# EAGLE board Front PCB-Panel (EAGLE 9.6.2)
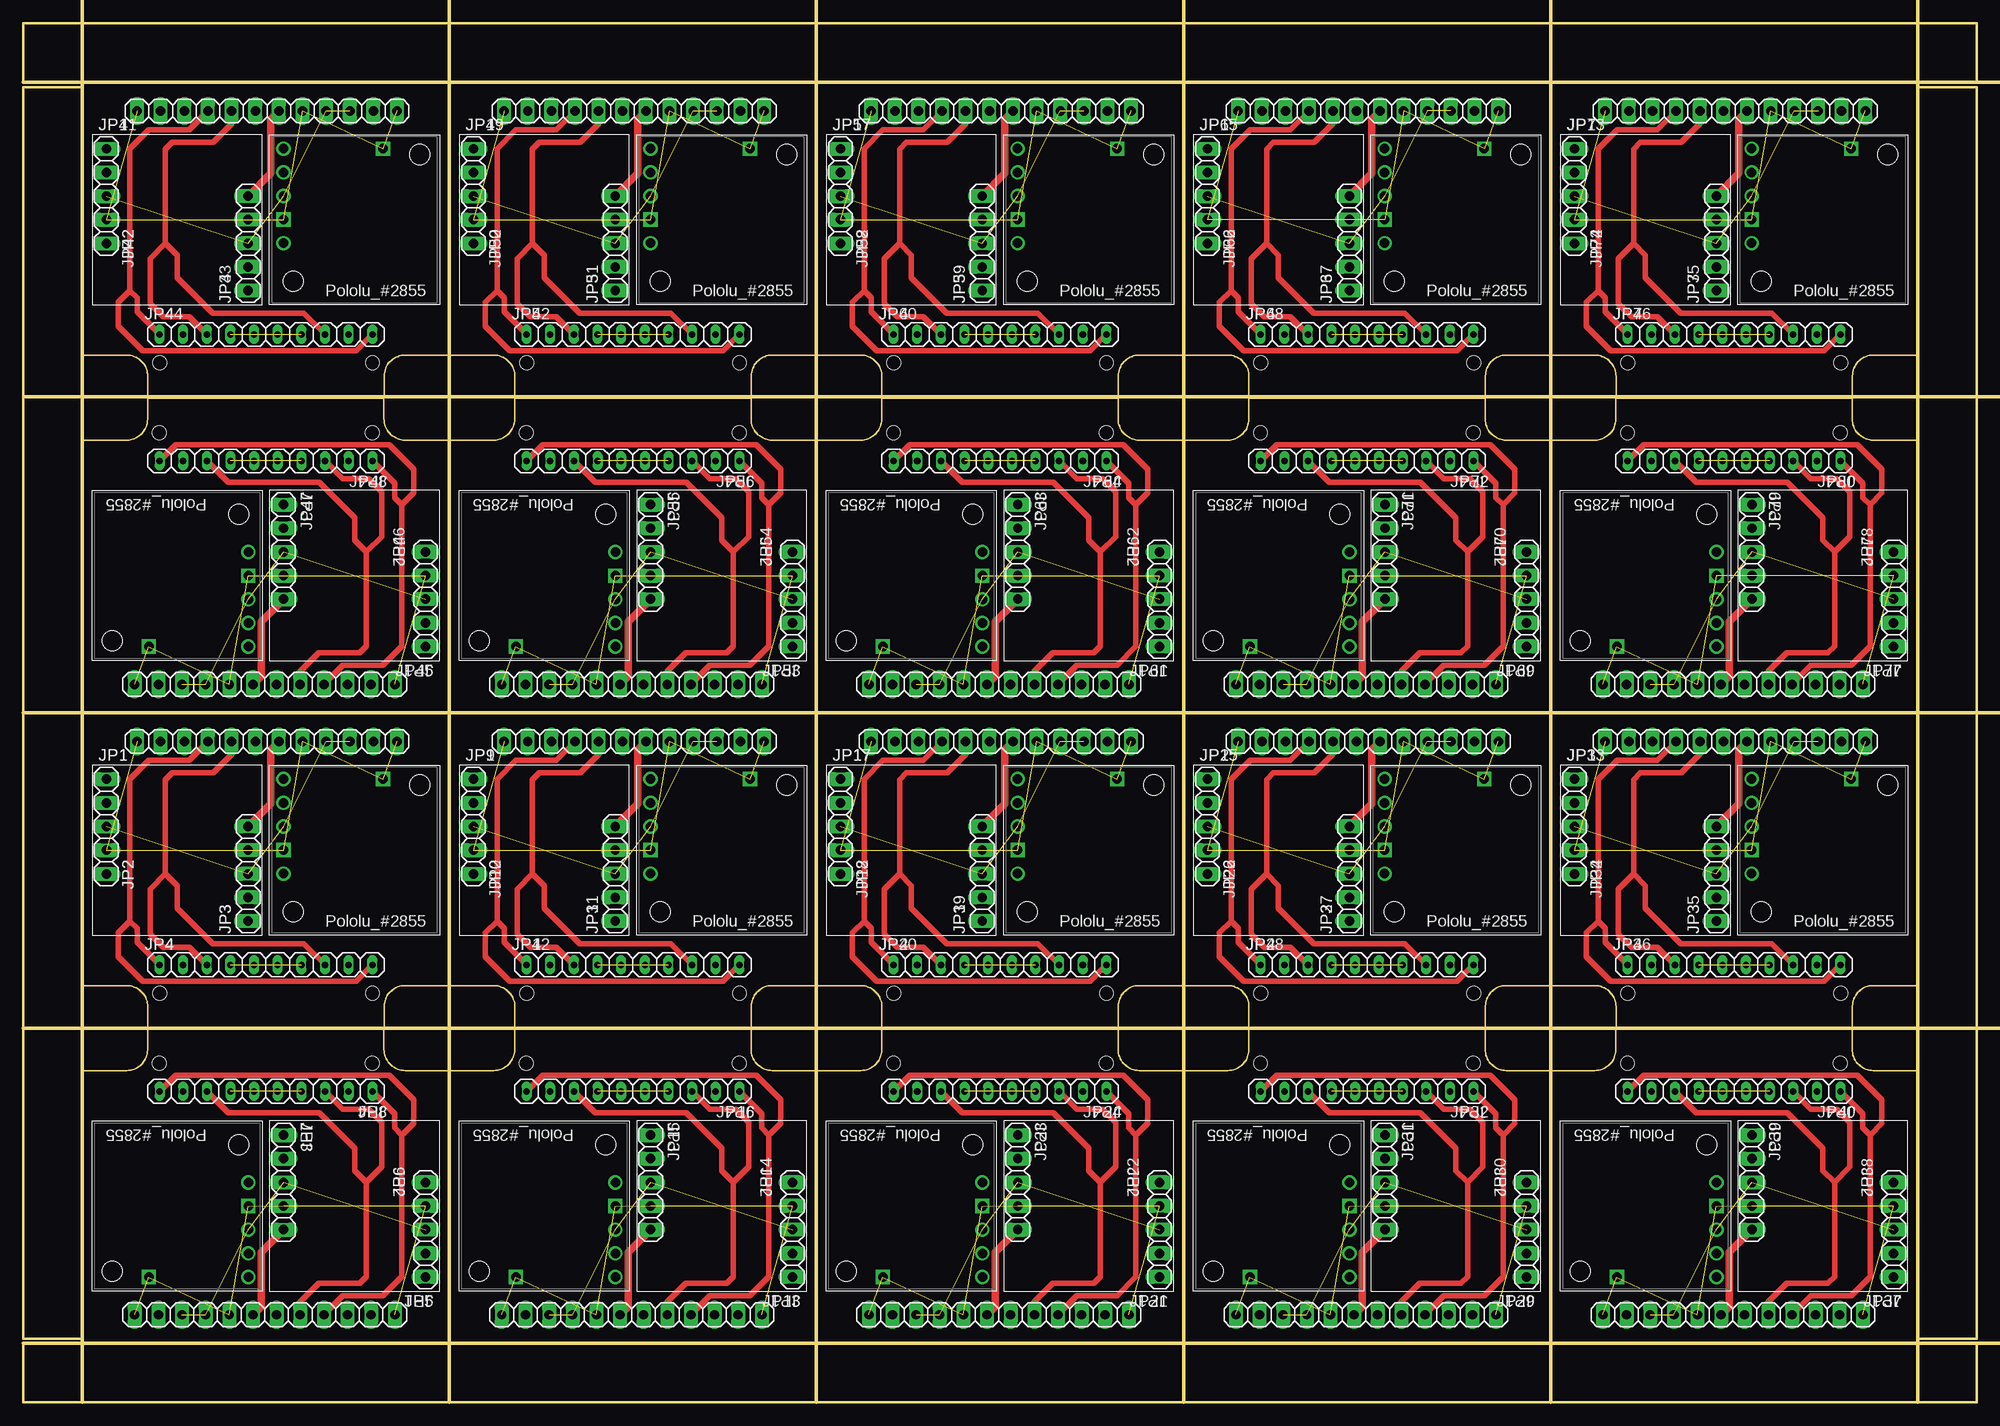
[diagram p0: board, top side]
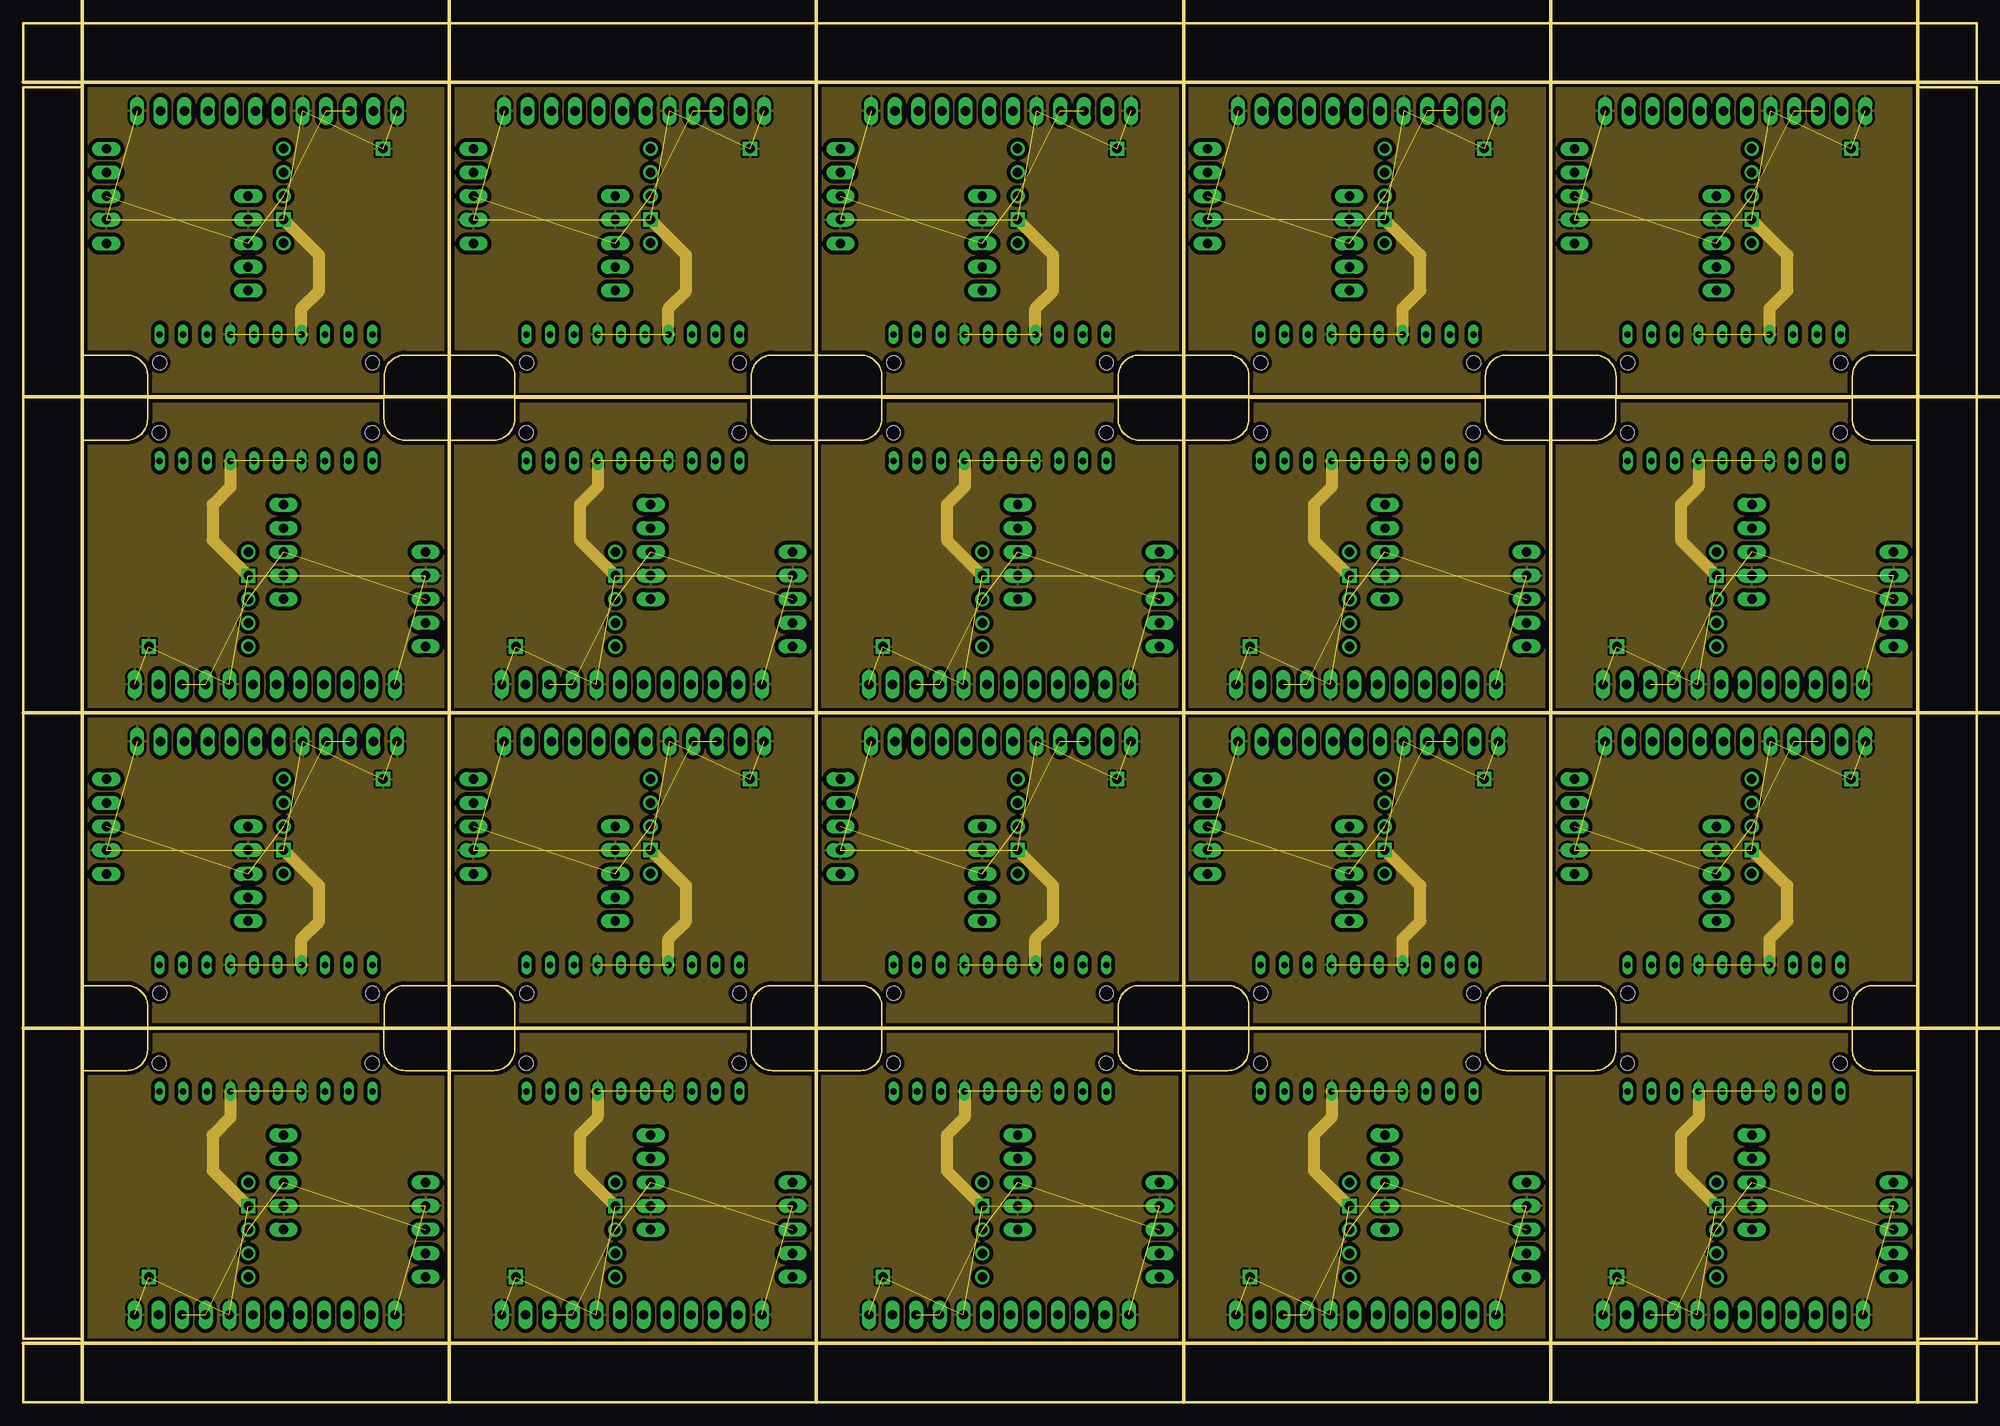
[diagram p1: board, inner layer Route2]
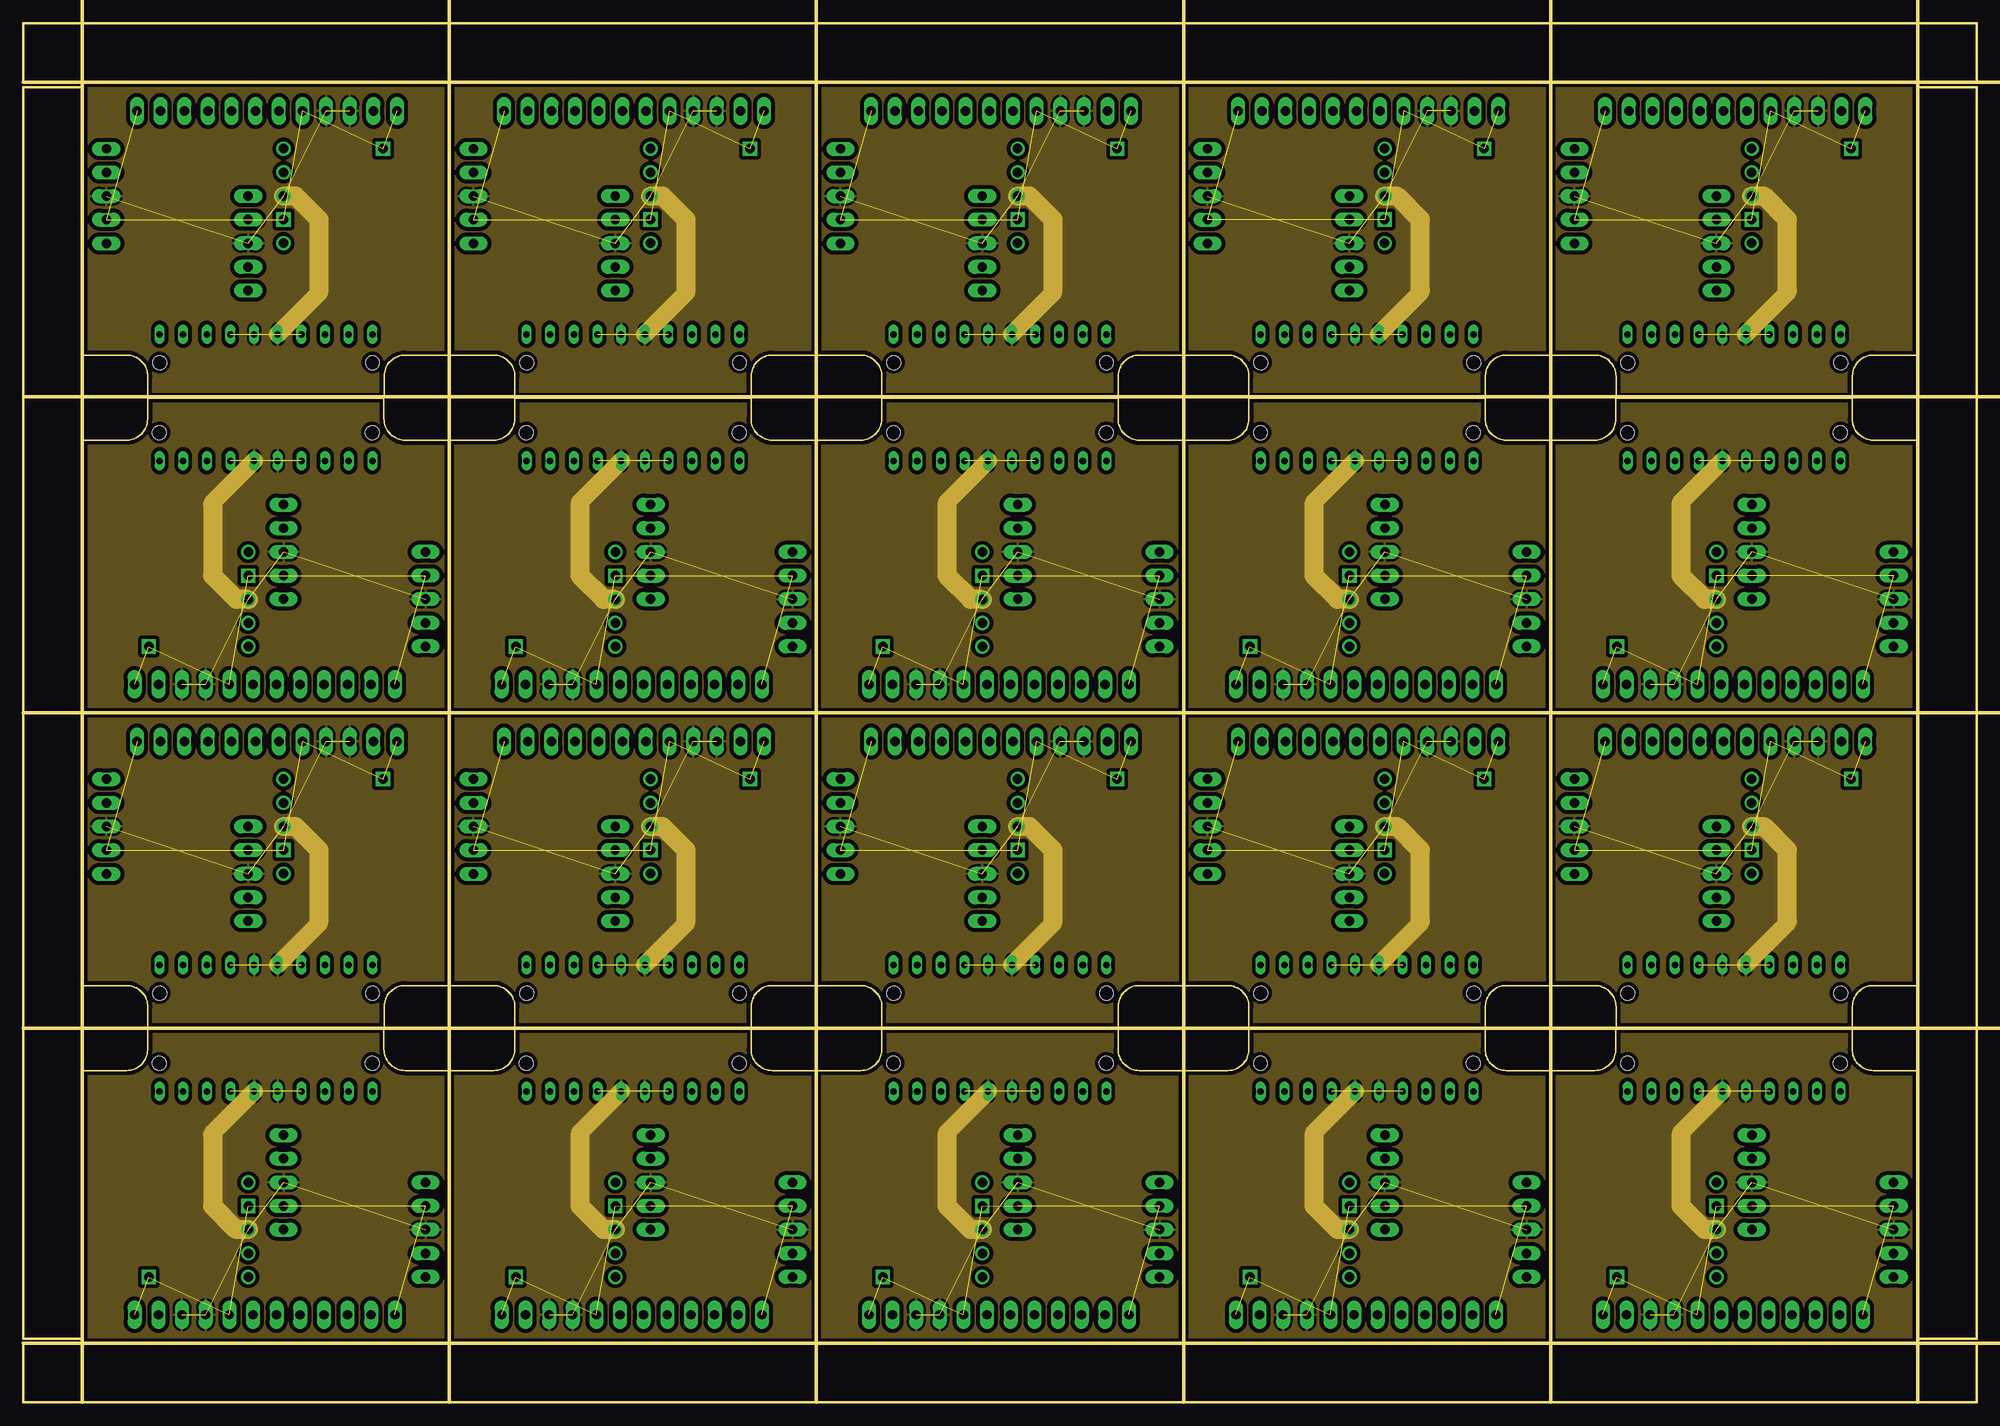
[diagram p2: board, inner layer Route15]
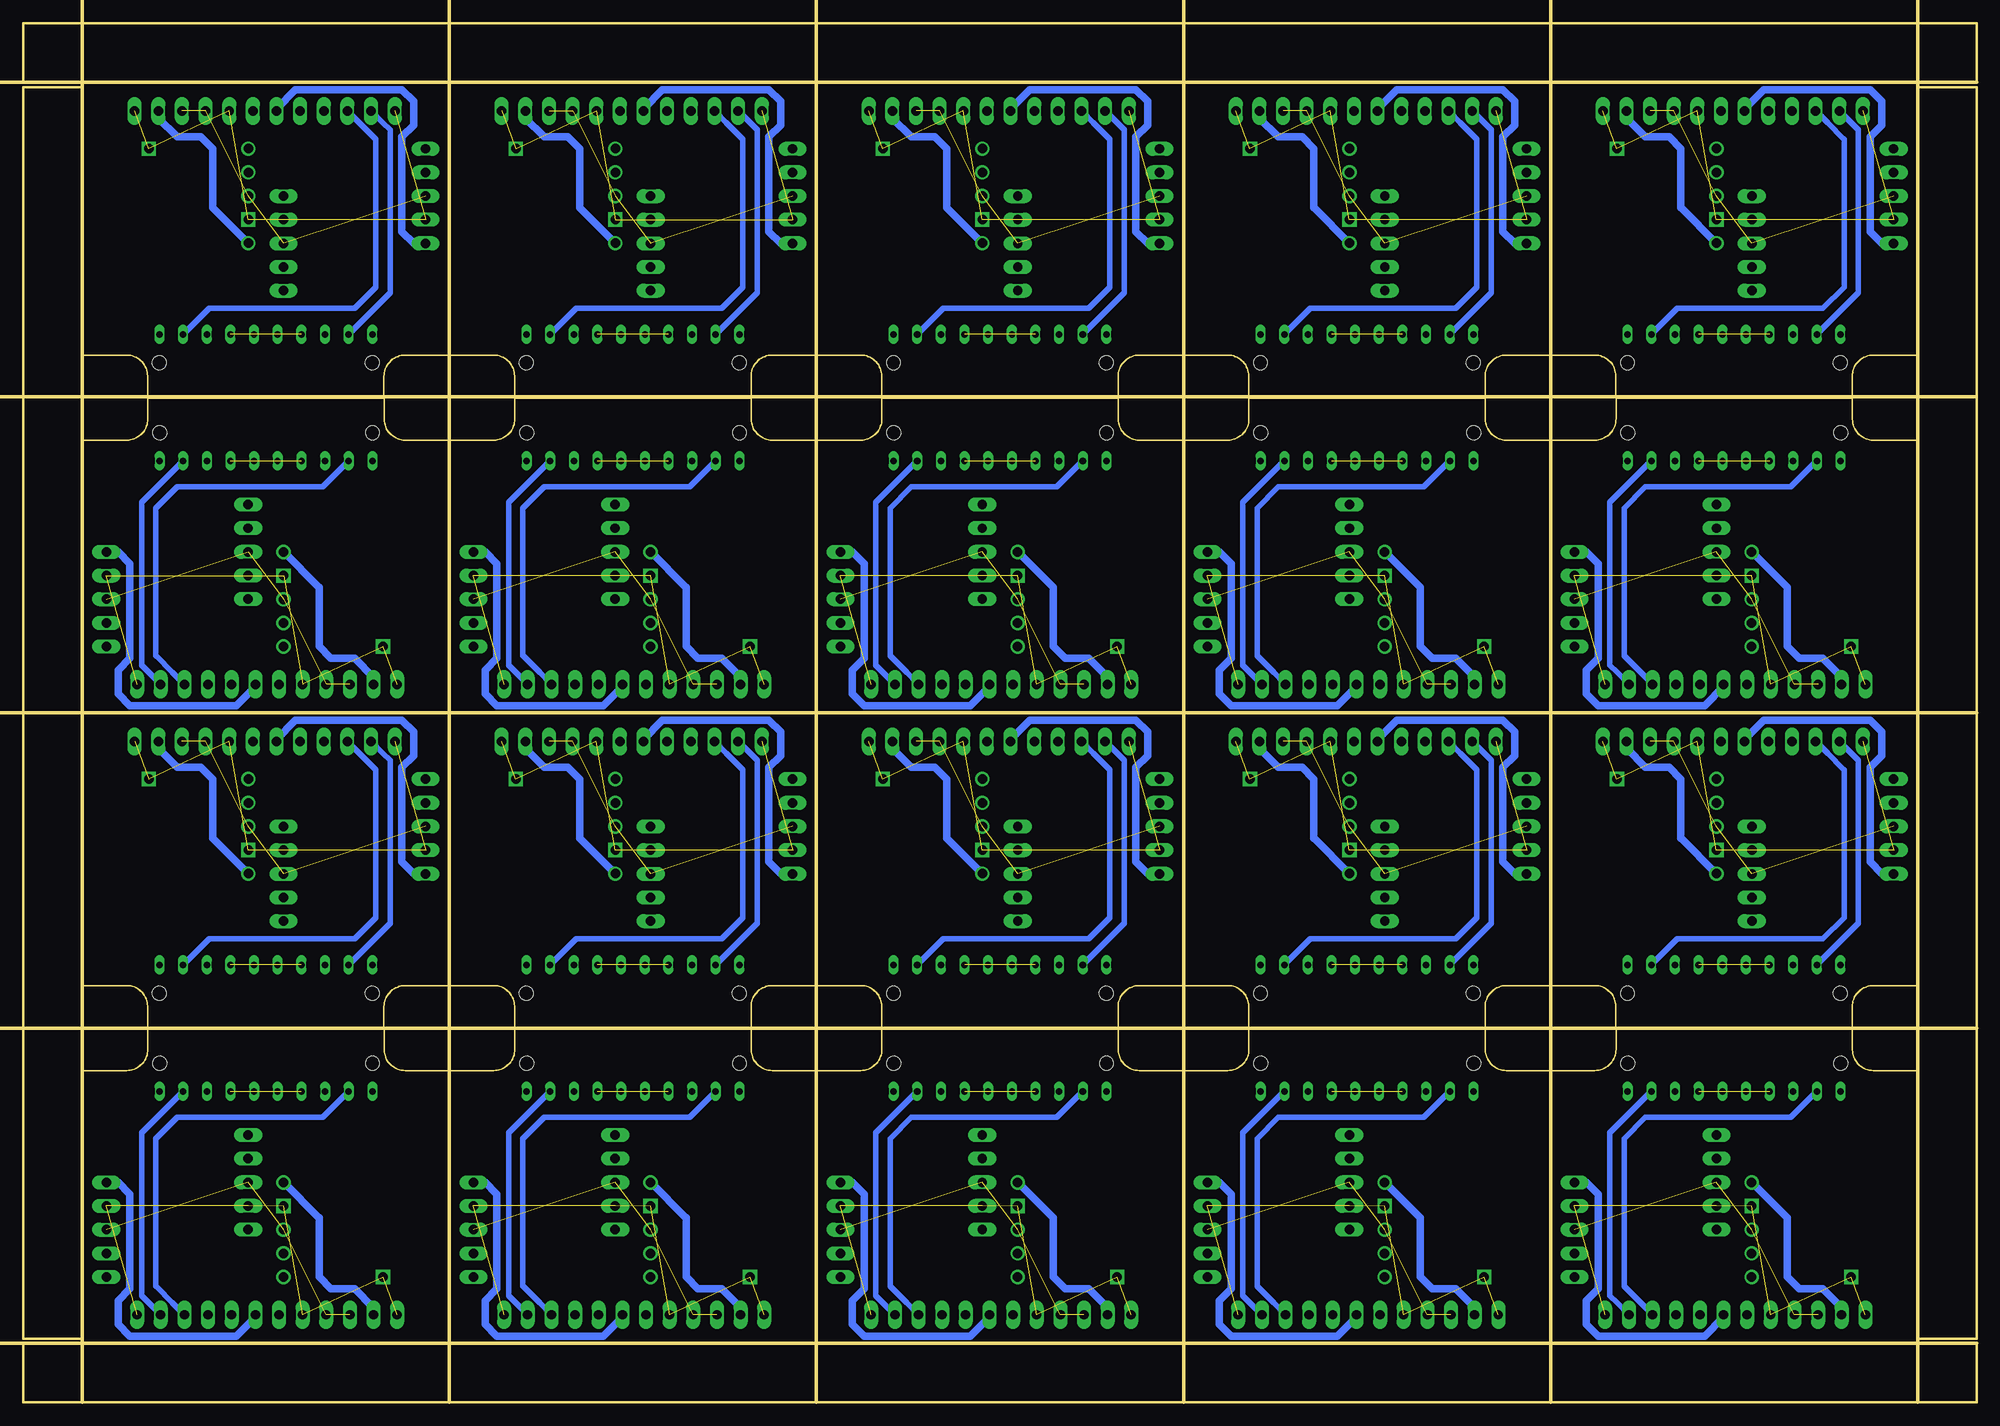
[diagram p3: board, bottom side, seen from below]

Size 209.85 x 148.15 mm. Coordinates in mm from the lower left corner, seen from the top.
Outline: 216 segments
Copper layers 1*2*15*16: Top 0.035mm / dielectric 0.171mm / Route2 0.0178mm / dielectric 44mil / Route15 0.025mm / dielectric 0.171mm / Bottom 0.035mm
Design rules "Front PCB": minimum track width 5mil, minimum drill 0.2mm, track to track 6mil, track to pad 6mil, pad to pad 6mil, via to via 6mil, smd to smd 5mil, copper to edge 0.002540625mm, drill to drill 5mil, minimum pad ring 4mil, minimum via ring 4mil, stop-mask expansion 4mil, vias tented up to drill 0mil, thermal gap 10mil
Holes 1.5 mm at 14.65,43.97 37.51,43.97 37.48,36.45 14.62,36.45 54.08,43.97 76.94,43.97 76.91,36.45 54.05,36.45 93.51,43.97 116.37,43.97 116.34,36.45 93.48,36.45 132.94,43.97 155.8,43.97 155.77,36.45 132.91,36.45 172.37,43.97 195.23,43.97 195.2,36.45 172.34,36.45 14.65,111.7 37.51,111.7 37.48,104.18 14.62,104.18 54.08,111.7 76.94,111.7 76.91,104.18 54.05,104.18 93.51,111.7 116.37,111.7 116.34,104.18 93.48,104.18 132.94,111.7 155.8,111.7 155.77,104.18 132.91,104.18 172.37,111.7 195.23,111.7 195.2,104.18 172.34,104.18
Milling: 11 lines

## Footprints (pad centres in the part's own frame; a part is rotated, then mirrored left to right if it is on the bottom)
POLOLU_D24V22FX = drill 1.02: 1 -7.63,7.63; 2 -7.63,5.09; 3 -7.63,2.55; 5 -7.63,-2.53 | drill 1.02 square: 4 -7.63,0.01; 6 3.06,7.63
1X12 = drill 1.016 long: 1 -13.97,0; 2 -11.43,0; 3 -8.89,0; 4 -6.35,0; 5 -3.81,0; 6 -1.27,0; 7 1.27,0; 8 3.81,0; 9 6.35,0; 10 8.89,0; 11 11.43,0; 12 13.97,0
1X05 = drill 1.016 long: 1 -5.08,0; 2 -2.54,0; 3 0,0; 4 2.54,0; 5 5.08,0
1X10 = drill 0.7 long: P$1 -11.43,0; P$2 -8.89,0; P$3 -6.35,0; P$4 -3.81,0; P$5 -1.27,0; P$6 1.27,0; P$7 3.81,0; P$8 6.35,0; P$9 8.89,0; P$10 11.43,0

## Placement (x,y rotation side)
12V  POLOLU_D24V22FX  [POLOLU_D24V22FX]  35.59,59.33 0 top
12V1  POLOLU_D24V22FX  [POLOLU_D24V22FX]  16.54,21.1 180 top
12V2  POLOLU_D24V22FX  [POLOLU_D24V22FX]  75.02,59.33 0 top
12V3  POLOLU_D24V22FX  [POLOLU_D24V22FX]  55.97,21.1 180 top
12V4  POLOLU_D24V22FX  [POLOLU_D24V22FX]  114.45,59.33 0 top
12V5  POLOLU_D24V22FX  [POLOLU_D24V22FX]  95.4,21.1 180 top
12V6  POLOLU_D24V22FX  [POLOLU_D24V22FX]  153.88,59.33 0 top
12V7  POLOLU_D24V22FX  [POLOLU_D24V22FX]  134.83,21.1 180 top
12V8  POLOLU_D24V22FX  [POLOLU_D24V22FX]  193.31,59.33 0 top
12V9  POLOLU_D24V22FX  [POLOLU_D24V22FX]  174.26,21.1 180 top
12V10  POLOLU_D24V22FX  [POLOLU_D24V22FX]  35.59,127.05 0 top
12V11  POLOLU_D24V22FX  [POLOLU_D24V22FX]  16.54,88.83 180 top
12V12  POLOLU_D24V22FX  [POLOLU_D24V22FX]  75.02,127.05 0 top
12V13  POLOLU_D24V22FX  [POLOLU_D24V22FX]  55.97,88.83 180 top
12V14  POLOLU_D24V22FX  [POLOLU_D24V22FX]  114.45,127.05 0 top
12V15  POLOLU_D24V22FX  [POLOLU_D24V22FX]  95.4,88.83 180 top
12V16  POLOLU_D24V22FX  [POLOLU_D24V22FX]  153.88,127.05 0 top
12V17  POLOLU_D24V22FX  [POLOLU_D24V22FX]  134.83,88.83 180 top
12V18  POLOLU_D24V22FX  [POLOLU_D24V22FX]  193.31,127.05 0 top
12V19  POLOLU_D24V22FX  [POLOLU_D24V22FX]  174.26,88.83 180 top
JP1  [1X12]  26.19,71.01 0 top
JP2  [1X05]  8.92,61.87 270 top
JP3  [1X05]  24.16,56.79 90 top
JP4  1X10  [1X10]  26.07,47.01 0 top
JP5  [1X12]  25.94,9.42 180 top
JP6  [1X05]  43.21,18.56 90 top
JP7  [1X05]  27.97,23.64 270 top
JP8  1X10  [1X10]  26.07,33.42 180 top
JP9  [1X12]  65.62,71.01 0 top
JP10  [1X05]  48.35,61.87 270 top
JP11  [1X05]  63.59,56.79 90 top
JP12  1X10  [1X10]  65.5,47.01 0 top
JP13  [1X12]  65.37,9.42 180 top
JP14  [1X05]  82.64,18.56 90 top
JP15  [1X05]  67.4,23.64 270 top
JP16  1X10  [1X10]  65.5,33.42 180 top
JP17  [1X12]  105.05,71.01 0 top
JP18  [1X05]  87.78,61.87 270 top
JP19  [1X05]  103.02,56.79 90 top
JP20  1X10  [1X10]  104.92,47.01 0 top
JP21  [1X12]  104.8,9.42 180 top
JP22  [1X05]  122.07,18.56 90 top
JP23  [1X05]  106.83,23.64 270 top
JP24  1X10  [1X10]  104.92,33.42 180 top
JP25  [1X12]  144.48,71.01 0 top
JP26  [1X05]  127.21,61.87 270 top
JP27  [1X05]  142.45,56.79 90 top
JP28  1X10  [1X10]  144.36,47.01 0 top
JP29  [1X12]  144.23,9.42 180 top
JP30  [1X05]  161.5,18.56 90 top
JP31  [1X05]  146.26,23.64 270 top
JP32  1X10  [1X10]  144.36,33.42 180 top
JP33  [1X12]  183.91,71.01 0 top
JP34  [1X05]  166.64,61.87 270 top
JP35  [1X05]  181.88,56.79 90 top
JP36  1X10  [1X10]  183.78,47.01 0 top
JP37  [1X12]  183.66,9.42 180 top
JP38  [1X05]  200.93,18.56 90 top
JP39  [1X05]  185.69,23.64 270 top
JP40  1X10  [1X10]  183.78,33.42 180 top
JP41  [1X12]  26.19,138.74 0 top
JP42  [1X05]  8.92,129.59 270 top
JP43  [1X05]  24.16,124.51 90 top
JP44  1X10  [1X10]  26.07,114.73 0 top
JP45  [1X12]  25.94,77.14 180 top
JP46  [1X05]  43.21,86.29 90 top
JP47  [1X05]  27.97,91.37 270 top
JP48  1X10  [1X10]  26.07,101.15 180 top
JP49  [1X12]  65.62,138.74 0 top
JP50  [1X05]  48.35,129.59 270 top
JP51  [1X05]  63.59,124.51 90 top
JP52  1X10  [1X10]  65.5,114.73 0 top
JP53  [1X12]  65.37,77.14 180 top
JP54  [1X05]  82.64,86.29 90 top
JP55  [1X05]  67.4,91.37 270 top
JP56  1X10  [1X10]  65.5,101.15 180 top
JP57  [1X12]  105.05,138.74 0 top
JP58  [1X05]  87.78,129.59 270 top
JP59  [1X05]  103.02,124.51 90 top
JP60  1X10  [1X10]  104.92,114.73 0 top
JP61  [1X12]  104.8,77.14 180 top
JP62  [1X05]  122.07,86.29 90 top
JP63  [1X05]  106.83,91.37 270 top
JP64  1X10  [1X10]  104.92,101.15 180 top
JP65  [1X12]  144.48,138.74 0 top
JP66  [1X05]  127.21,129.59 270 top
JP67  [1X05]  142.45,124.51 90 top
JP68  1X10  [1X10]  144.36,114.73 0 top
JP69  [1X12]  144.23,77.14 180 top
JP70  [1X05]  161.5,86.29 90 top
JP71  [1X05]  146.26,91.37 270 top
JP72  1X10  [1X10]  144.36,101.15 180 top
JP73  [1X12]  183.91,138.74 0 top
JP74  [1X05]  166.64,129.59 270 top
JP75  [1X05]  181.88,124.51 90 top
JP76  1X10  [1X10]  183.78,114.73 0 top
JP77  [1X12]  183.66,77.14 180 top
JP78  [1X05]  200.93,86.29 90 top
JP79  [1X05]  185.69,91.37 270 top
JP80  1X10  [1X10]  183.78,101.15 180 top

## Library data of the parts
12V 12V1-12V19 = POLOLU_D24V22FX
JP1-JP3 JP5-JP7 JP9-JP11 JP13-JP15 JP17-JP19 JP21-JP23 JP25-JP27 JP29-JP31 JP33-JP35 JP37-JP39 JP41-JP43 JP45-JP47 JP49-JP51 JP53-JP55 JP57-JP59 JP61-JP63 JP65-JP67 JP69-JP71 JP73-JP75 JP77-JP79 = pinhead
JP4 JP8 JP12 JP16 JP20 JP24 JP28 JP32 JP36 JP40 JP44 JP48 JP52 JP56 JP60 JP64 JP68 JP72 JP76 JP80 = Pinheads 2.54mm 0.7diameter

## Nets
5V [2A]: JP1.7 JP3.5
5V1 [2A]: JP5.7 JP7.5
5V2 [2A]: JP9.7 JP11.5
5V3 [2A]: JP13.7 JP15.5
5V4 [2A]: JP17.7 JP19.5
5V5 [2A]: JP21.7 JP23.5
5V6 [2A]: JP25.7 JP27.5
5V7 [2A]: JP29.7 JP31.5
5V8 [2A]: JP33.7 JP35.5
5V9 [2A]: JP37.7 JP39.5
5V10 [2A]: JP41.7 JP43.5
5V11 [2A]: JP45.7 JP47.5
5V12 [2A]: JP49.7 JP51.5
5V13 [2A]: JP53.7 JP55.5
5V14 [2A]: JP57.7 JP59.5
5V15 [2A]: JP61.7 JP63.5
5V16 [2A]: JP65.7 JP67.5
5V17 [2A]: JP69.7 JP71.5
5V18 [2A]: JP73.7 JP75.5
5V19 [2A]: JP77.7 JP79.5
6V [1A]: JP1.6 JP2.5
6V1 [1A]: JP5.6 JP6.5
6V2 [1A]: JP9.6 JP10.5
6V3 [1A]: JP13.6 JP14.5
6V4 [1A]: JP17.6 JP18.5
6V5 [1A]: JP21.6 JP22.5
6V6 [1A]: JP25.6 JP26.5
6V7 [1A]: JP29.6 JP30.5
6V8 [1A]: JP33.6 JP34.5
6V9 [1A]: JP37.6 JP38.5
6V10 [1A]: JP41.6 JP42.5
6V11 [1A]: JP45.6 JP46.5
6V12 [1A]: JP49.6 JP50.5
6V13 [1A]: JP53.6 JP54.5
6V14 [1A]: JP57.6 JP58.5
6V15 [1A]: JP61.6 JP62.5
6V16 [1A]: JP65.6 JP66.5
6V17 [1A]: JP69.6 JP70.5
6V18 [1A]: JP73.6 JP74.5
6V19 [1A]: JP77.6 JP78.5
12V [1A]: 12V.5 JP1.11
12V1 [1A]: 12V1.5 JP5.11
12V2 [1A]: 12V2.5 JP9.11
12V3 [1A]: 12V3.5 JP13.11
12V4 [1A]: 12V4.5 JP17.11
12V5 [1A]: 12V5.5 JP21.11
12V6 [1A]: 12V6.5 JP25.11
12V7 [1A]: 12V7.5 JP29.11
12V8 [1A]: 12V8.5 JP33.11
12V9 [1A]: 12V9.5 JP37.11
12V10 [1A]: 12V10.5 JP41.11
12V11 [1A]: 12V11.5 JP45.11
12V12 [1A]: 12V12.5 JP49.11
12V13 [1A]: 12V13.5 JP53.11
12V14 [1A]: 12V14.5 JP57.11
12V15 [1A]: 12V15.5 JP61.11
12V16 [1A]: 12V16.5 JP65.11
12V17 [1A]: 12V17.5 JP69.11
12V18 [1A]: 12V18.5 JP73.11
12V19 [1A]: 12V19.5 JP77.11
24V [3A]: 12V.3 JP1.9 JP1.10 JP2.3 JP3.3 JP4.P$5 JP4.P$6
24V1 [3A]: 12V1.3 JP5.9 JP5.10 JP6.3 JP7.3 JP8.P$5 JP8.P$6
24V2 [3A]: 12V2.3 JP9.9 JP9.10 JP10.3 JP11.3 JP12.P$5 JP12.P$6
24V3 [3A]: 12V3.3 JP13.9 JP13.10 JP14.3 JP15.3 JP16.P$5 JP16.P$6
24V4 [3A]: 12V4.3 JP17.9 JP17.10 JP18.3 JP19.3 JP20.P$5 JP20.P$6
24V5 [3A]: 12V5.3 JP21.9 JP21.10 JP22.3 JP23.3 JP24.P$5 JP24.P$6
24V6 [3A]: 12V6.3 JP25.9 JP25.10 JP26.3 JP27.3 JP28.P$5 JP28.P$6
24V7 [3A]: 12V7.3 JP29.9 JP29.10 JP30.3 JP31.3 JP32.P$5 JP32.P$6
24V8 [3A]: 12V8.3 JP33.9 JP33.10 JP34.3 JP35.3 JP36.P$5 JP36.P$6
24V9 [3A]: 12V9.3 JP37.9 JP37.10 JP38.3 JP39.3 JP40.P$5 JP40.P$6
24V10 [3A]: 12V10.3 JP41.9 JP41.10 JP42.3 JP43.3 JP44.P$5 JP44.P$6
24V11 [3A]: 12V11.3 JP45.9 JP45.10 JP46.3 JP47.3 JP48.P$5 JP48.P$6
24V12 [3A]: 12V12.3 JP49.9 JP49.10 JP50.3 JP51.3 JP52.P$5 JP52.P$6
24V13 [3A]: 12V13.3 JP53.9 JP53.10 JP54.3 JP55.3 JP56.P$5 JP56.P$6
24V14 [3A]: 12V14.3 JP57.9 JP57.10 JP58.3 JP59.3 JP60.P$5 JP60.P$6
24V15 [3A]: 12V15.3 JP61.9 JP61.10 JP62.3 JP63.3 JP64.P$5 JP64.P$6
24V16 [3A]: 12V16.3 JP65.9 JP65.10 JP66.3 JP67.3 JP68.P$5 JP68.P$6
24V17 [3A]: 12V17.3 JP69.9 JP69.10 JP70.3 JP71.3 JP72.P$5 JP72.P$6
24V18 [3A]: 12V18.3 JP73.9 JP73.10 JP74.3 JP75.3 JP76.P$5 JP76.P$6
24V19 [3A]: 12V19.3 JP77.9 JP77.10 JP78.3 JP79.3 JP80.P$5 JP80.P$6
DIR#1: JP1.2 JP4.P$2
DIR#2: JP1.3 JP4.P$9
DIR#3: JP5.2 JP8.P$2
DIR#4: JP5.3 JP8.P$9
DIR#5: JP9.2 JP12.P$2
DIR#6: JP9.3 JP12.P$9
DIR#7: JP13.2 JP16.P$2
DIR#8: JP13.3 JP16.P$9
DIR#9: JP17.2 JP20.P$2
DIR#10: JP17.3 JP20.P$9
DIR#11: JP21.2 JP24.P$2
DIR#12: JP21.3 JP24.P$9
DIR#13: JP25.2 JP28.P$2
DIR#14: JP25.3 JP28.P$9
DIR#15: JP29.2 JP32.P$2
DIR#16: JP29.3 JP32.P$9
DIR#17: JP33.2 JP36.P$2
DIR#18: JP33.3 JP36.P$9
DIR#19: JP37.2 JP40.P$2
DIR#20: JP37.3 JP40.P$9
DIR#21: JP41.2 JP44.P$2
DIR#22: JP41.3 JP44.P$9
DIR#23: JP45.2 JP48.P$2
DIR#24: JP45.3 JP48.P$9
DIR#25: JP49.2 JP52.P$2
DIR#26: JP49.3 JP52.P$9
DIR#27: JP53.2 JP56.P$2
DIR#28: JP53.3 JP56.P$9
DIR#29: JP57.2 JP60.P$2
DIR#30: JP57.3 JP60.P$9
DIR#31: JP61.2 JP64.P$2
DIR#32: JP61.3 JP64.P$9
DIR#33: JP65.2 JP68.P$2
DIR#34: JP65.3 JP68.P$9
DIR#35: JP69.2 JP72.P$2
DIR#36: JP69.3 JP72.P$9
DIR#37: JP73.2 JP76.P$2
DIR#38: JP73.3 JP76.P$9
DIR#39: JP77.2 JP80.P$2
DIR#40: JP77.3 JP80.P$9
GND: 12V.4 12V.6 JP1.1 JP1.8 JP1.12 JP2.4 JP3.4 JP4.P$4 JP4.P$7
GND1: 12V1.4 12V1.6 JP5.1 JP5.8 JP5.12 JP6.4 JP7.4 JP8.P$4 JP8.P$7
GND2: 12V2.4 12V2.6 JP9.1 JP9.8 JP9.12 JP10.4 JP11.4 JP12.P$4 JP12.P$7
GND3: 12V3.4 12V3.6 JP13.1 JP13.8 JP13.12 JP14.4 JP15.4 JP16.P$4 JP16.P$7
GND4: 12V4.4 12V4.6 JP17.1 JP17.8 JP17.12 JP18.4 JP19.4 JP20.P$4 JP20.P$7
GND5: 12V5.4 12V5.6 JP21.1 JP21.8 JP21.12 JP22.4 JP23.4 JP24.P$4 JP24.P$7
GND6: 12V6.4 12V6.6 JP25.1 JP25.8 JP25.12 JP26.4 JP27.4 JP28.P$4 JP28.P$7
GND7: 12V7.4 12V7.6 JP29.1 JP29.8 JP29.12 JP30.4 JP31.4 JP32.P$4 JP32.P$7
GND8: 12V8.4 12V8.6 JP33.1 JP33.8 JP33.12 JP34.4 JP35.4 JP36.P$4 JP36.P$7
GND9: 12V9.4 12V9.6 JP37.1 JP37.8 JP37.12 JP38.4 JP39.4 JP40.P$4 JP40.P$7
GND10: 12V10.4 12V10.6 JP41.1 JP41.8 JP41.12 JP42.4 JP43.4 JP44.P$4 JP44.P$7
GND11: 12V11.4 12V11.6 JP45.1 JP45.8 JP45.12 JP46.4 JP47.4 JP48.P$4 JP48.P$7
GND12: 12V12.4 12V12.6 JP49.1 JP49.8 JP49.12 JP50.4 JP51.4 JP52.P$4 JP52.P$7
GND13: 12V13.4 12V13.6 JP53.1 JP53.8 JP53.12 JP54.4 JP55.4 JP56.P$4 JP56.P$7
GND14: 12V14.4 12V14.6 JP57.1 JP57.8 JP57.12 JP58.4 JP59.4 JP60.P$4 JP60.P$7
GND15: 12V15.4 12V15.6 JP61.1 JP61.8 JP61.12 JP62.4 JP63.4 JP64.P$4 JP64.P$7
GND16: 12V16.4 12V16.6 JP65.1 JP65.8 JP65.12 JP66.4 JP67.4 JP68.P$4 JP68.P$7
GND17: 12V17.4 12V17.6 JP69.1 JP69.8 JP69.12 JP70.4 JP71.4 JP72.P$4 JP72.P$7
GND18: 12V18.4 12V18.6 JP73.1 JP73.8 JP73.12 JP74.4 JP75.4 JP76.P$4 JP76.P$7
GND19: 12V19.4 12V19.6 JP77.1 JP77.8 JP77.12 JP78.4 JP79.4 JP80.P$4 JP80.P$7
HAIVE_ID: JP1.5 JP4.P$3 JP4.P$8
HAIVE_ID1: JP5.5 JP8.P$3 JP8.P$8
HAIVE_ID2: JP9.5 JP12.P$3 JP12.P$8
HAIVE_ID3: JP13.5 JP16.P$3 JP16.P$8
HAIVE_ID4: JP17.5 JP20.P$3 JP20.P$8
HAIVE_ID5: JP21.5 JP24.P$3 JP24.P$8
HAIVE_ID6: JP25.5 JP28.P$3 JP28.P$8
HAIVE_ID7: JP29.5 JP32.P$3 JP32.P$8
HAIVE_ID8: JP33.5 JP36.P$3 JP36.P$8
HAIVE_ID9: JP37.5 JP40.P$3 JP40.P$8
HAIVE_ID10: JP41.5 JP44.P$3 JP44.P$8
HAIVE_ID11: JP45.5 JP48.P$3 JP48.P$8
HAIVE_ID12: JP49.5 JP52.P$3 JP52.P$8
HAIVE_ID13: JP53.5 JP56.P$3 JP56.P$8
HAIVE_ID14: JP57.5 JP60.P$3 JP60.P$8
HAIVE_ID15: JP61.5 JP64.P$3 JP64.P$8
HAIVE_ID16: JP65.5 JP68.P$3 JP68.P$8
HAIVE_ID17: JP69.5 JP72.P$3 JP72.P$8
HAIVE_ID18: JP73.5 JP76.P$3 JP76.P$8
HAIVE_ID19: JP77.5 JP80.P$3 JP80.P$8
SLOT_ID: JP1.4 JP4.P$1 JP4.P$10
SLOT_ID1: JP5.4 JP8.P$1 JP8.P$10
SLOT_ID2: JP9.4 JP12.P$1 JP12.P$10
SLOT_ID3: JP13.4 JP16.P$1 JP16.P$10
SLOT_ID4: JP17.4 JP20.P$1 JP20.P$10
SLOT_ID5: JP21.4 JP24.P$1 JP24.P$10
SLOT_ID6: JP25.4 JP28.P$1 JP28.P$10
SLOT_ID7: JP29.4 JP32.P$1 JP32.P$10
SLOT_ID8: JP33.4 JP36.P$1 JP36.P$10
SLOT_ID9: JP37.4 JP40.P$1 JP40.P$10
SLOT_ID10: JP41.4 JP44.P$1 JP44.P$10
SLOT_ID11: JP45.4 JP48.P$1 JP48.P$10
SLOT_ID12: JP49.4 JP52.P$1 JP52.P$10
SLOT_ID13: JP53.4 JP56.P$1 JP56.P$10
SLOT_ID14: JP57.4 JP60.P$1 JP60.P$10
SLOT_ID15: JP61.4 JP64.P$1 JP64.P$10
SLOT_ID16: JP65.4 JP68.P$1 JP68.P$10
SLOT_ID17: JP69.4 JP72.P$1 JP72.P$10
SLOT_ID18: JP73.4 JP76.P$1 JP76.P$10
SLOT_ID19: JP77.4 JP80.P$1 JP80.P$10

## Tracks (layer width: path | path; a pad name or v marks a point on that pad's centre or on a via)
5V
  Top 0.813: JP3.5 26.59,64.3 26.59,70.14 JP1.7
5V1
  Top 0.813: JP7.5 25.54,16.13 25.54,10.29 JP5.7
5V2
  Top 0.813: JP11.5 66.02,64.3 66.02,70.14 JP9.7
5V3
  Top 0.813: JP15.5 64.97,16.13 64.97,10.29 JP13.7
5V4
  Top 0.813: JP19.5 105.45,64.3 105.45,70.14 JP17.7
5V5
  Top 0.813: JP23.5 104.4,16.13 104.4,10.29 JP21.7
5V6
  Top 0.813: JP27.5 144.88,64.3 144.88,70.14 JP25.7
5V7
  Top 0.813: JP31.5 143.83,16.13 143.83,10.29 JP29.7
5V8
  Top 0.813: JP35.5 184.31,64.3 184.31,70.14 JP33.7
5V9
  Top 0.813: JP39.5 183.26,16.13 183.26,10.29 JP37.7
5V10
  Top 0.813: JP43.5 26.59,132.02 26.59,137.86 JP41.7
5V11
  Top 0.813: JP47.5 25.54,83.86 25.54,78.02 JP45.7
5V12
  Top 0.813: JP51.5 66.02,132.02 66.02,137.86 JP49.7
5V13
  Top 0.813: JP55.5 64.97,83.86 64.97,78.02 JP53.7
5V14
  Top 0.813: JP59.5 105.45,132.02 105.45,137.86 JP57.7
5V15
  Top 0.813: JP63.5 104.4,83.86 104.4,78.02 JP61.7
5V16
  Top 0.813: JP67.5 144.88,132.02 144.88,137.86 JP65.7
5V17
  Top 0.813: JP71.5 143.83,83.86 143.83,78.02 JP69.7
5V18
  Top 0.813: JP75.5 184.31,132.02 184.31,137.86 JP73.7
5V19
  Top 0.813: JP79.5 183.26,83.86 183.26,78.02 JP77.7
6V
  Bottom 0.813: JP1.6 24.92,71.27 22.89,73.3 11.46,73.3 10.19,72.03 10.19,69.49 11.46,68.22 11.46,58.06 10.19,56.79 JP2.5
6V1
  Bottom 0.813: JP5.6 27.21,9.16 29.24,7.13 40.67,7.13 41.94,8.4 41.94,10.94 40.67,12.21 40.67,22.37 41.94,23.64 JP6.5
6V2
  Bottom 0.813: JP9.6 64.35,71.27 62.32,73.3 50.89,73.3 49.62,72.03 49.62,69.49 50.89,68.22 50.89,58.06 49.62,56.79 JP10.5
6V3
  Bottom 0.813: JP13.6 66.64,9.16 68.67,7.13 80.1,7.13 81.37,8.4 81.37,10.94 80.1,12.21 80.1,22.37 81.37,23.64 JP14.5
6V4
  Bottom 0.813: JP17.6 103.78,71.27 101.75,73.3 90.32,73.3 89.05,72.03 89.05,69.49 90.32,68.22 90.32,58.06 89.05,56.79 JP18.5
6V5
  Bottom 0.813: JP21.6 106.07,9.16 108.1,7.13 119.53,7.13 120.8,8.4 120.8,10.94 119.53,12.21 119.53,22.37 120.8,23.64 JP22.5
6V6
  Bottom 0.813: JP25.6 143.21,71.27 141.18,73.3 129.75,73.3 128.48,72.03 128.48,69.49 129.75,68.22 129.75,58.06 128.48,56.79 JP26.5
6V7
  Bottom 0.813: JP29.6 145.5,9.16 147.53,7.13 158.96,7.13 160.23,8.4 160.23,10.94 158.96,12.21 158.96,22.37 160.23,23.64 JP30.5
6V8
  Bottom 0.813: JP33.6 182.64,71.27 180.61,73.3 169.18,73.3 167.91,72.03 167.91,69.49 169.18,68.22 169.18,58.06 167.91,56.79 JP34.5
6V9
  Bottom 0.813: JP37.6 184.93,9.16 186.96,7.13 198.39,7.13 199.66,8.4 199.66,10.94 198.39,12.21 198.39,22.37 199.66,23.64 JP38.5
6V10
  Bottom 0.813: JP41.6 24.92,138.99 22.89,141.02 11.46,141.02 10.19,139.75 10.19,137.21 11.46,135.94 11.46,125.78 10.19,124.51 JP42.5
6V11
  Bottom 0.813: JP45.6 27.21,76.89 29.24,74.86 40.67,74.86 41.94,76.13 41.94,78.67 40.67,79.94 40.67,90.1 41.94,91.37 JP46.5
6V12
  Bottom 0.813: JP49.6 64.35,138.99 62.32,141.02 50.89,141.02 49.62,139.75 49.62,137.21 50.89,135.94 50.89,125.78 49.62,124.51 JP50.5
6V13
  Bottom 0.813: JP53.6 66.64,76.89 68.67,74.86 80.1,74.86 81.37,76.13 81.37,78.67 80.1,79.94 80.1,90.1 81.37,91.37 JP54.5
6V14
  Bottom 0.813: JP57.6 103.78,138.99 101.75,141.02 90.32,141.02 89.05,139.75 89.05,137.21 90.32,135.94 90.32,125.78 89.05,124.51 JP58.5
6V15
  Bottom 0.813: JP61.6 106.07,76.89 108.1,74.86 119.53,74.86 120.8,76.13 120.8,78.67 119.53,79.94 119.53,90.1 120.8,91.37 JP62.5
6V16
  Bottom 0.813: JP65.6 143.21,138.99 141.18,141.02 129.75,141.02 128.48,139.75 128.48,137.21 129.75,135.94 129.75,125.78 128.48,124.51 JP66.5
6V17
  Bottom 0.813: JP69.6 145.5,76.89 147.53,74.86 158.96,74.86 160.23,76.13 160.23,78.67 158.96,79.94 158.96,90.1 160.23,91.37 JP70.5
6V18
  Bottom 0.813: JP73.6 182.64,138.99 180.61,141.02 169.18,141.02 167.91,139.75 167.91,137.21 169.18,135.94 169.18,125.78 167.91,124.51 JP74.5
6V19
  Bottom 0.813: JP77.6 184.93,76.89 186.96,74.86 198.39,74.86 199.66,76.13 199.66,78.67 198.39,79.94 198.39,90.1 199.66,91.37 JP78.5
12V
  Bottom 0.813: 12V.5 31.76,60.6 31.78,60.6 31.78,66.95 33.05,68.22 35.59,68.22 37.62,70.25 JP1.11
12V1
  Bottom 0.813: 12V1.5 20.37,19.83 20.35,19.83 20.35,13.48 19.08,12.21 16.54,12.21 14.51,10.18 JP5.11
12V2
  Bottom 0.813: 12V2.5 71.19,60.6 71.21,60.6 71.21,66.95 72.48,68.22 75.02,68.22 77.05,70.25 JP9.11
12V3
  Bottom 0.813: 12V3.5 59.8,19.83 59.78,19.83 59.78,13.48 58.51,12.21 55.97,12.21 53.94,10.18 JP13.11
12V4
  Bottom 0.813: 12V4.5 110.62,60.6 110.64,60.6 110.64,66.95 111.91,68.22 114.45,68.22 116.48,70.25 JP17.11
12V5
  Bottom 0.813: 12V5.5 99.23,19.83 99.21,19.83 99.21,13.48 97.94,12.21 95.4,12.21 93.37,10.18 JP21.11
12V6
  Bottom 0.813: 12V6.5 150.05,60.6 150.07,60.6 150.07,66.95 151.34,68.22 153.88,68.22 155.91,70.25 JP25.11
12V7
  Bottom 0.813: 12V7.5 138.66,19.83 138.64,19.83 138.64,13.48 137.37,12.21 134.83,12.21 132.8,10.18 JP29.11
12V8
  Bottom 0.813: 12V8.5 189.48,60.6 189.5,60.6 189.5,66.95 190.77,68.22 193.31,68.22 195.34,70.25 JP33.11
12V9
  Bottom 0.813: 12V9.5 178.09,19.83 178.07,19.83 178.07,13.48 176.8,12.21 174.26,12.21 172.23,10.18 JP37.11
12V10
  Bottom 0.813: 12V10.5 31.76,128.32 31.78,128.32 31.78,134.67 33.05,135.94 35.59,135.94 37.62,137.97 JP41.11
12V11
  Bottom 0.813: 12V11.5 20.37,87.56 20.35,87.56 20.35,81.21 19.08,79.94 16.54,79.94 14.51,77.9 JP45.11
12V12
  Bottom 0.813: 12V12.5 71.19,128.32 71.21,128.32 71.21,134.67 72.48,135.94 75.02,135.94 77.05,137.97 JP49.11
12V13
  Bottom 0.813: 12V13.5 59.8,87.56 59.78,87.56 59.78,81.21 58.51,79.94 55.97,79.94 53.94,77.9 JP53.11
12V14
  Bottom 0.813: 12V14.5 110.62,128.32 110.64,128.32 110.64,134.67 111.91,135.94 114.45,135.94 116.48,137.97 JP57.11
12V15
  Bottom 0.813: 12V15.5 99.23,87.56 99.21,87.56 99.21,81.21 97.94,79.94 95.4,79.94 93.37,77.9 JP61.11
12V16
  Bottom 0.813: 12V16.5 150.05,128.32 150.07,128.32 150.07,134.67 151.34,135.94 153.88,135.94 155.91,137.97 JP65.11
12V17
  Bottom 0.813: 12V17.5 138.66,87.56 138.64,87.56 138.64,81.21 137.37,79.94 134.83,79.94 132.8,77.9 JP69.11
12V18
  Bottom 0.813: 12V18.5 189.48,128.32 189.5,128.32 189.5,134.67 190.77,135.94 193.31,135.94 195.34,137.97 JP73.11
12V19
  Bottom 0.813: 12V19.5 178.09,87.56 178.07,87.56 178.07,81.21 176.8,79.94 174.26,79.94 172.23,77.9 JP77.11
24V  (5 unrouted)
  Route15 1.905: JP4.P$6 31.78,51.45 31.78,51.71
  Route15 2.032: 12V.3 29.23,61.88 31.78,59.33 31.78,51.71
  pour Route15 (isolate 0.406): 6.38,74.06 45.75,74.06 45.75,44.34 41.8,44.34 arc90 39.15,41.68 39.15,40.28 12.98,40.28 12.98,41.68 arc90 10.33,44.34 6.38,44.34
24V1  (5 unrouted)
  Route15 1.905: JP8.P$6 20.35,28.97 20.35,28.72
  Route15 2.032: 12V1.3 22.9,18.55 20.35,21.1 20.35,28.72
  pour Route15 (isolate 0.406): 45.75,6.37 6.38,6.37 6.38,36.09 10.33,36.09 arc90 12.98,38.74 12.98,40.15 39.15,40.15 39.15,38.74 arc90 41.8,36.09 45.75,36.09
24V2  (5 unrouted)
  Route15 1.905: JP12.P$6 71.21,51.45 71.21,51.71
  Route15 2.032: 12V2.3 68.66,61.88 71.21,59.33 71.21,51.71
  pour Route15 (isolate 0.406): 45.81,74.06 85.18,74.06 85.18,44.34 81.24,44.34 arc90 78.58,41.68 78.58,40.28 52.42,40.28 52.42,41.68 arc90 49.76,44.34 45.81,44.34
24V3  (5 unrouted)
  Route15 1.905: JP16.P$6 59.78,28.97 59.78,28.72
  Route15 2.032: 12V3.3 62.33,18.55 59.78,21.1 59.78,28.72
  pour Route15 (isolate 0.406): 85.18,6.37 45.81,6.37 45.81,36.09 49.76,36.09 arc90 52.42,38.74 52.42,40.15 78.58,40.15 78.58,38.74 arc90 81.24,36.09 85.18,36.09
24V4  (5 unrouted)
  Route15 1.905: JP20.P$6 110.64,51.45 110.64,51.71
  Route15 2.032: 12V4.3 108.09,61.88 110.64,59.33 110.64,51.71
  pour Route15 (isolate 0.406): 85.24,74.06 124.61,74.06 124.61,44.34 120.66,44.34 arc90 118.01,41.68 118.01,40.28 91.84,40.28 91.84,41.68 arc90 89.19,44.34 85.24,44.34
24V5  (5 unrouted)
  Route15 1.905: JP24.P$6 99.21,28.97 99.21,28.72
  Route15 2.032: 12V5.3 101.76,18.55 99.21,21.1 99.21,28.72
  pour Route15 (isolate 0.406): 124.61,6.37 85.24,6.37 85.24,36.09 89.19,36.09 arc90 91.84,38.74 91.84,40.15 118.01,40.15 118.01,38.74 arc90 120.66,36.09 124.61,36.09
24V6  (5 unrouted)
  Route15 1.905: JP28.P$6 150.07,51.45 150.07,51.71
  Route15 2.032: 12V6.3 147.52,61.88 150.07,59.33 150.07,51.71
  pour Route15 (isolate 0.406): 124.67,74.06 164.04,74.06 164.04,44.34 160.09,44.34 arc90 157.44,41.68 157.44,40.28 131.27,40.28 131.27,41.68 arc90 128.62,44.34 124.67,44.34
24V7  (5 unrouted)
  Route15 1.905: JP32.P$6 138.64,28.97 138.64,28.72
  Route15 2.032: 12V7.3 141.19,18.55 138.64,21.1 138.64,28.72
  pour Route15 (isolate 0.406): 164.04,6.37 124.67,6.37 124.67,36.09 128.62,36.09 arc90 131.27,38.74 131.27,40.15 157.44,40.15 157.44,38.74 arc90 160.09,36.09 164.04,36.09
24V8  (5 unrouted)
  Route15 1.905: JP36.P$6 189.5,51.45 189.5,51.71
  Route15 2.032: 12V8.3 186.95,61.88 189.5,59.33 189.5,51.71
  pour Route15 (isolate 0.406): 164.1,74.06 203.47,74.06 203.47,44.34 199.52,44.34 arc90 196.87,41.68 196.87,40.28 170.7,40.28 170.7,41.68 arc90 168.05,44.34 164.1,44.34
24V9  (5 unrouted)
  Route15 1.905: JP40.P$6 178.07,28.97 178.07,28.72
  Route15 2.032: 12V9.3 180.62,18.55 178.07,21.1 178.07,28.72
  pour Route15 (isolate 0.406): 203.47,6.37 164.1,6.37 164.1,36.09 168.05,36.09 arc90 170.7,38.74 170.7,40.15 196.87,40.15 196.87,38.74 arc90 199.52,36.09 203.47,36.09
24V10  (5 unrouted)
  Route15 1.905: JP44.P$6 31.78,119.18 31.78,119.43
  Route15 2.032: 12V10.3 29.23,129.6 31.78,127.05 31.78,119.43
  pour Route15 (isolate 0.406): 6.38,141.79 45.75,141.79 45.75,112.07 41.8,112.07 arc90 39.15,109.41 39.15,108 12.98,108 12.98,109.41 arc90 10.33,112.07 6.38,112.07
24V11  (5 unrouted)
  Route15 1.905: JP48.P$6 20.35,96.7 20.35,96.45
  Route15 2.032: 12V11.3 22.9,86.28 20.35,88.83 20.35,96.45
  pour Route15 (isolate 0.406): 45.75,74.09 6.38,74.09 6.38,103.81 10.33,103.81 arc90 12.98,106.47 12.98,107.88 39.15,107.88 39.15,106.47 arc90 41.8,103.81 45.75,103.81
24V12  (5 unrouted)
  Route15 1.905: JP52.P$6 71.21,119.18 71.21,119.43
  Route15 2.032: 12V12.3 68.66,129.6 71.21,127.05 71.21,119.43
  pour Route15 (isolate 0.406): 45.81,141.79 85.18,141.79 85.18,112.07 81.24,112.07 arc90 78.58,109.41 78.58,108 52.42,108 52.42,109.41 arc90 49.76,112.07 45.81,112.07
24V13  (5 unrouted)
  Route15 1.905: JP56.P$6 59.78,96.7 59.78,96.45
  Route15 2.032: 12V13.3 62.33,86.28 59.78,88.83 59.78,96.45
  pour Route15 (isolate 0.406): 85.18,74.09 45.81,74.09 45.81,103.81 49.76,103.81 arc90 52.42,106.47 52.42,107.88 78.58,107.88 78.58,106.47 arc90 81.24,103.81 85.18,103.81
24V14  (5 unrouted)
  Route15 1.905: JP60.P$6 110.64,119.18 110.64,119.43
  Route15 2.032: 12V14.3 108.09,129.6 110.64,127.05 110.64,119.43
  pour Route15 (isolate 0.406): 85.24,141.79 124.61,141.79 124.61,112.07 120.66,112.07 arc90 118.01,109.41 118.01,108 91.84,108 91.84,109.41 arc90 89.19,112.07 85.24,112.07
24V15  (5 unrouted)
  Route15 1.905: JP64.P$6 99.21,96.7 99.21,96.45
  Route15 2.032: 12V15.3 101.76,86.28 99.21,88.83 99.21,96.45
  pour Route15 (isolate 0.406): 124.61,74.09 85.24,74.09 85.24,103.81 89.19,103.81 arc90 91.84,106.47 91.84,107.88 118.01,107.88 118.01,106.47 arc90 120.66,103.81 124.61,103.81
24V16  (5 unrouted)
  Route15 1.905: JP68.P$6 150.07,119.18 150.07,119.43
  Route15 2.032: 12V16.3 147.52,129.6 150.07,127.05 150.07,119.43
  pour Route15 (isolate 0.406): 124.67,141.79 164.04,141.79 164.04,112.07 160.09,112.07 arc90 157.44,109.41 157.44,108 131.27,108 131.27,109.41 arc90 128.62,112.07 124.67,112.07
24V17  (5 unrouted)
  Route15 1.905: JP72.P$6 138.64,96.7 138.64,96.45
  Route15 2.032: 12V17.3 141.19,86.28 138.64,88.83 138.64,96.45
  pour Route15 (isolate 0.406): 164.04,74.09 124.67,74.09 124.67,103.81 128.62,103.81 arc90 131.27,106.47 131.27,107.88 157.44,107.88 157.44,106.47 arc90 160.09,103.81 164.04,103.81
24V18  (5 unrouted)
  Route15 1.905: JP76.P$6 189.5,119.18 189.5,119.43
  Route15 2.032: 12V18.3 186.95,129.6 189.5,127.05 189.5,119.43
  pour Route15 (isolate 0.406): 164.1,141.79 203.47,141.79 203.47,112.07 199.52,112.07 arc90 196.87,109.41 196.87,108 170.7,108 170.7,109.41 arc90 168.05,112.07 164.1,112.07
24V19  (5 unrouted)
  Route15 1.905: JP80.P$6 178.07,96.7 178.07,96.45
  Route15 2.032: 12V19.3 180.62,86.28 178.07,88.83 178.07,96.45
  pour Route15 (isolate 0.406): 203.47,74.09 164.1,74.09 164.1,103.81 168.05,103.81 arc90 170.7,106.47 170.7,107.88 196.87,107.88 196.87,106.47 arc90 199.52,103.81 203.47,103.81
DIR#1
  Bottom 0.61: JP1.2 13.49,69.74 13.49,69.72 12.73,68.97 12.73,51.45 JP4.P$2
DIR#2
  Bottom 0.61: JP1.3 16.03,69.74 16.03,69.72 14.27,67.96 14.25,67.96 14.25,52.09 16.54,49.8 31.78,49.8 32.16,49.8 JP4.P$9
DIR#3
  Bottom 0.61: JP5.2 38.64,10.69 38.64,10.7 39.4,11.46 39.4,28.97 JP8.P$2
DIR#4
  Bottom 0.61: JP5.3 36.1,10.69 36.1,10.7 37.86,12.46 37.88,12.46 37.88,28.34 35.59,30.62 19.97,30.62 JP8.P$9
DIR#5
  Bottom 0.61: JP9.2 52.92,69.74 52.92,69.72 52.16,68.97 52.16,51.45 JP12.P$2
DIR#6
  Bottom 0.61: JP9.3 55.46,69.74 55.46,69.72 53.7,67.96 53.69,67.96 53.69,52.09 55.97,49.8 71.21,49.8 71.59,49.8 JP12.P$9
DIR#7
  Bottom 0.61: JP13.2 78.07,10.69 78.07,10.7 78.83,11.46 78.83,28.97 JP16.P$2
DIR#8
  Bottom 0.61: JP13.3 75.53,10.69 75.53,10.7 77.29,12.46 77.31,12.46 77.31,28.34 75.02,30.62 59.4,30.62 JP16.P$9
DIR#9
  Bottom 0.61: JP17.2 92.35,69.74 92.35,69.72 91.59,68.97 91.59,51.45 JP20.P$2
DIR#10
  Bottom 0.61: JP17.3 94.89,69.74 94.89,69.72 93.13,67.96 93.11,67.96 93.11,52.09 95.4,49.8 110.64,49.8 111.02,49.8 JP20.P$9
DIR#11
  Bottom 0.61: JP21.2 117.5,10.69 117.5,10.7 118.26,11.46 118.26,28.97 JP24.P$2
DIR#12
  Bottom 0.61: JP21.3 114.96,10.69 114.96,10.7 116.72,12.46 116.74,12.46 116.74,28.34 114.45,30.62 98.83,30.62 JP24.P$9
DIR#13
  Bottom 0.61: JP25.2 131.78,69.74 131.78,69.72 131.02,68.97 131.02,51.45 JP28.P$2
DIR#14
  Bottom 0.61: JP25.3 134.32,69.74 134.32,69.72 132.56,67.96 132.54,67.96 132.54,52.09 134.83,49.8 150.07,49.8 150.45,49.8 JP28.P$9
DIR#15
  Bottom 0.61: JP29.2 156.93,10.69 156.93,10.7 157.69,11.46 157.69,28.97 JP32.P$2
DIR#16
  Bottom 0.61: JP29.3 154.39,10.69 154.39,10.7 156.15,12.46 156.17,12.46 156.17,28.34 153.88,30.62 138.26,30.62 JP32.P$9
DIR#17
  Bottom 0.61: JP33.2 171.21,69.74 171.21,69.72 170.45,68.97 170.45,51.45 JP36.P$2
DIR#18
  Bottom 0.61: JP33.3 173.75,69.74 173.75,69.72 171.99,67.96 171.97,67.96 171.97,52.09 174.26,49.8 189.5,49.8 189.88,49.8 JP36.P$9
DIR#19
  Bottom 0.61: JP37.2 196.36,10.69 196.36,10.7 197.12,11.46 197.12,28.97 JP40.P$2
DIR#20
  Bottom 0.61: JP37.3 193.82,10.69 193.82,10.7 195.58,12.46 195.59,12.46 195.59,28.34 193.31,30.62 177.69,30.62 JP40.P$9
DIR#21
  Bottom 0.61: JP41.2 13.49,137.46 13.49,137.45 12.73,136.69 12.73,119.18 JP44.P$2
DIR#22
  Bottom 0.61: JP41.3 16.03,137.46 16.03,137.45 14.27,135.69 14.25,135.69 14.25,119.81 16.54,117.53 31.78,117.53 32.16,117.53 JP44.P$9
DIR#23
  Bottom 0.61: JP45.2 38.64,78.42 38.64,78.43 39.4,79.19 39.4,96.7 JP48.P$2
DIR#24
  Bottom 0.61: JP45.3 36.1,78.42 36.1,78.43 37.86,80.19 37.88,80.19 37.88,96.06 35.59,98.35 19.97,98.35 JP48.P$9
DIR#25
  Bottom 0.61: JP49.2 52.92,137.46 52.92,137.45 52.16,136.69 52.16,119.18 JP52.P$2
DIR#26
  Bottom 0.61: JP49.3 55.46,137.46 55.46,137.45 53.7,135.69 53.69,135.69 53.69,119.81 55.97,117.53 71.21,117.53 71.59,117.53 JP52.P$9
DIR#27
  Bottom 0.61: JP53.2 78.07,78.42 78.07,78.43 78.83,79.19 78.83,96.7 JP56.P$2
DIR#28
  Bottom 0.61: JP53.3 75.53,78.42 75.53,78.43 77.29,80.19 77.31,80.19 77.31,96.06 75.02,98.35 59.4,98.35 JP56.P$9
DIR#29
  Bottom 0.61: JP57.2 92.35,137.46 92.35,137.45 91.59,136.69 91.59,119.18 JP60.P$2
DIR#30
  Bottom 0.61: JP57.3 94.89,137.46 94.89,137.45 93.13,135.69 93.11,135.69 93.11,119.81 95.4,117.53 110.64,117.53 111.02,117.53 JP60.P$9
DIR#31
  Bottom 0.61: JP61.2 117.5,78.42 117.5,78.43 118.26,79.19 118.26,96.7 JP64.P$2
DIR#32
  Bottom 0.61: JP61.3 114.96,78.42 114.96,78.43 116.72,80.19 116.74,80.19 116.74,96.06 114.45,98.35 98.83,98.35 JP64.P$9
DIR#33
  Bottom 0.61: JP65.2 131.78,137.46 131.78,137.45 131.02,136.69 131.02,119.18 JP68.P$2
DIR#34
  Bottom 0.61: JP65.3 134.32,137.46 134.32,137.45 132.56,135.69 132.54,135.69 132.54,119.81 134.83,117.53 150.07,117.53 150.45,117.53 JP68.P$9
DIR#35
  Bottom 0.61: JP69.2 156.93,78.42 156.93,78.43 157.69,79.19 157.69,96.7 JP72.P$2
DIR#36
  Bottom 0.61: JP69.3 154.39,78.42 154.39,78.43 156.15,80.19 156.17,80.19 156.17,96.06 153.88,98.35 138.26,98.35 JP72.P$9
DIR#37
  Bottom 0.61: JP73.2 171.21,137.46 171.21,137.45 170.45,136.69 170.45,119.18 JP76.P$2
DIR#38
  Bottom 0.61: JP73.3 173.75,137.46 173.75,137.45 171.99,135.69 171.97,135.69 171.97,119.81 174.26,117.53 189.5,117.53 189.88,117.53 JP76.P$9
DIR#39
  Bottom 0.61: JP77.2 196.36,78.42 196.36,78.43 197.12,79.19 197.12,96.7 JP80.P$2
DIR#40
  Bottom 0.61: JP77.3 193.82,78.42 193.82,78.43 195.58,80.19 195.59,80.19 195.59,96.06 193.31,98.35 177.69,98.35 JP80.P$9
GND  (7 unrouted)
  Route2 1.27: 12V.4 31.78,55.52 31.78,51.71 29.88,49.8 JP4.P$7
  pour Route2 (isolate 0.406): 6.38,74.06 45.75,74.06 45.75,44.34 42,44.34 arc90 39.02,41.36 39.02,40.28 13.24,40.28 13.24,41.06 arc90 9.96,44.34 6.38,44.34
GND1  (7 unrouted)
  Route2 1.27: 12V1.4 20.35,24.91 20.35,28.72 22.25,30.62 JP8.P$7
  pour Route2 (isolate 0.406): 45.75,6.37 6.38,6.37 6.38,36.09 10.13,36.09 arc90 13.11,39.07 13.11,40.15 38.89,40.15 38.89,39.36 arc90 42.17,36.09 45.75,36.09
GND2  (7 unrouted)
  Route2 1.27: 12V2.4 71.21,55.52 71.21,51.71 69.31,49.8 JP12.P$7
  pour Route2 (isolate 0.406): 45.81,74.06 85.18,74.06 85.18,44.34 81.43,44.34 arc90 78.45,41.36 78.45,40.28 52.67,40.28 52.67,41.06 arc90 49.39,44.34 45.81,44.34
GND3  (7 unrouted)
  Route2 1.27: 12V3.4 59.78,24.91 59.78,28.72 61.69,30.62 JP16.P$7
  pour Route2 (isolate 0.406): 85.18,6.37 45.81,6.37 45.81,36.09 49.56,36.09 arc90 52.54,39.07 52.54,40.15 78.32,40.15 78.32,39.36 arc90 81.6,36.09 85.18,36.09
GND4  (7 unrouted)
  Route2 1.27: 12V4.4 110.64,55.52 110.64,51.71 108.73,49.8 JP20.P$7
  pour Route2 (isolate 0.406): 85.24,74.06 124.61,74.06 124.61,44.34 120.86,44.34 arc90 117.88,41.36 117.88,40.28 92.1,40.28 92.1,41.06 arc90 88.82,44.34 85.24,44.34
GND5  (7 unrouted)
  Route2 1.27: 12V5.4 99.21,24.91 99.21,28.72 101.11,30.62 JP24.P$7
  pour Route2 (isolate 0.406): 124.61,6.37 85.24,6.37 85.24,36.09 88.99,36.09 arc90 91.97,39.07 91.97,40.15 117.75,40.15 117.75,39.36 arc90 121.03,36.09 124.61,36.09
GND6  (7 unrouted)
  Route2 1.27: 12V6.4 150.07,55.52 150.07,51.71 148.17,49.8 JP28.P$7
  pour Route2 (isolate 0.406): 124.67,74.06 164.04,74.06 164.04,44.34 160.29,44.34 arc90 157.31,41.36 157.31,40.28 131.53,40.28 131.53,41.06 arc90 128.25,44.34 124.67,44.34
GND7  (7 unrouted)
  Route2 1.27: 12V7.4 138.64,24.91 138.64,28.72 140.55,30.62 JP32.P$7
  pour Route2 (isolate 0.406): 164.04,6.37 124.67,6.37 124.67,36.09 128.42,36.09 arc90 131.4,39.07 131.4,40.15 157.18,40.15 157.18,39.36 arc90 160.46,36.09 164.04,36.09
GND8  (7 unrouted)
  Route2 1.27: 12V8.4 189.5,55.52 189.5,51.71 187.59,49.8 JP36.P$7
  pour Route2 (isolate 0.406): 164.1,74.06 203.47,74.06 203.47,44.34 199.72,44.34 arc90 196.74,41.36 196.74,40.28 170.96,40.28 170.96,41.06 arc90 167.68,44.34 164.1,44.34
GND9  (7 unrouted)
  Route2 1.27: 12V9.4 178.07,24.91 178.07,28.72 179.97,30.62 JP40.P$7
  pour Route2 (isolate 0.406): 203.47,6.37 164.1,6.37 164.1,36.09 167.85,36.09 arc90 170.83,39.07 170.83,40.15 196.61,40.15 196.61,39.36 arc90 199.89,36.09 203.47,36.09
GND10  (7 unrouted)
  Route2 1.27: 12V10.4 31.78,123.24 31.78,119.43 29.88,117.53 JP44.P$7
  pour Route2 (isolate 0.406): 6.38,141.79 45.75,141.79 45.75,112.07 42,112.07 arc90 39.02,109.08 39.02,108 13.24,108 13.24,108.79 arc90 9.96,112.07 6.38,112.07
GND11  (7 unrouted)
  Route2 1.27: 12V11.4 20.35,92.64 20.35,96.45 22.25,98.35 JP48.P$7
  pour Route2 (isolate 0.406): 45.75,74.09 6.38,74.09 6.38,103.81 10.13,103.81 arc90 13.11,106.79 13.11,107.88 38.89,107.88 38.89,107.09 arc90 42.17,103.81 45.75,103.81
GND12  (7 unrouted)
  Route2 1.27: 12V12.4 71.21,123.24 71.21,119.43 69.31,117.53 JP52.P$7
  pour Route2 (isolate 0.406): 45.81,141.79 85.18,141.79 85.18,112.07 81.43,112.07 arc90 78.45,109.08 78.45,108 52.67,108 52.67,108.79 arc90 49.39,112.07 45.81,112.07
GND13  (7 unrouted)
  Route2 1.27: 12V13.4 59.78,92.64 59.78,96.45 61.69,98.35 JP56.P$7
  pour Route2 (isolate 0.406): 85.18,74.09 45.81,74.09 45.81,103.81 49.56,103.81 arc90 52.54,106.79 52.54,107.88 78.32,107.88 78.32,107.09 arc90 81.6,103.81 85.18,103.81
GND14  (7 unrouted)
  Route2 1.27: 12V14.4 110.64,123.24 110.64,119.43 108.73,117.53 JP60.P$7
  pour Route2 (isolate 0.406): 85.24,141.79 124.61,141.79 124.61,112.07 120.86,112.07 arc90 117.88,109.08 117.88,108 92.1,108 92.1,108.79 arc90 88.82,112.07 85.24,112.07
GND15  (7 unrouted)
  Route2 1.27: 12V15.4 99.21,92.64 99.21,96.45 101.11,98.35 JP64.P$7
  pour Route2 (isolate 0.406): 124.61,74.09 85.24,74.09 85.24,103.81 88.99,103.81 arc90 91.97,106.79 91.97,107.88 117.75,107.88 117.75,107.09 arc90 121.03,103.81 124.61,103.81
GND16  (7 unrouted)
  Route2 1.27: 12V16.4 150.07,123.24 150.07,119.43 148.17,117.53 JP68.P$7
  pour Route2 (isolate 0.406): 124.67,141.79 164.04,141.79 164.04,112.07 160.29,112.07 arc90 157.31,109.08 157.31,108 131.53,108 131.53,108.79 arc90 128.25,112.07 124.67,112.07
GND17  (7 unrouted)
  Route2 1.27: 12V17.4 138.64,92.64 138.64,96.45 140.55,98.35 JP72.P$7
  pour Route2 (isolate 0.406): 164.04,74.09 124.67,74.09 124.67,103.81 128.42,103.81 arc90 131.4,106.79 131.4,107.88 157.18,107.88 157.18,107.09 arc90 160.46,103.81 164.04,103.81
GND18  (7 unrouted)
  Route2 1.27: 12V18.4 189.5,123.24 189.5,119.43 187.59,117.53 JP76.P$7
  pour Route2 (isolate 0.406): 164.1,141.79 203.47,141.79 203.47,112.07 199.72,112.07 arc90 196.74,109.08 196.74,108 170.96,108 170.96,108.79 arc90 167.68,112.07 164.1,112.07
GND19  (7 unrouted)
  Route2 1.27: 12V19.4 178.07,92.64 178.07,96.45 179.97,98.35 JP80.P$7
  pour Route2 (isolate 0.406): 203.47,74.09 164.1,74.09 164.1,103.81 167.85,103.81 arc90 170.83,106.79 170.83,107.88 196.61,107.88 196.61,107.09 arc90 199.89,103.81 203.47,103.81
HAIVE_ID
  Top 0.61: JP1.5 22.38,69.61 20.4,67.63 16,67.63 15.27,66.9 15.27,56.79 | 15.27,56.79 16.54,55.52 16.54,53.1 20.35,49.29 30.13,49.29 JP4.P$8 | 15.27,56.79 13.62,55.14 13.62,50.31 14.38,49.55 14.51,49.42 15.02,48.91 17.81,48.91 JP4.P$3
HAIVE_ID1
  Top 0.61: JP5.5 29.75,10.81 31.73,12.8 36.13,12.8 36.86,13.52 36.86,23.64 | 36.86,23.64 35.59,24.91 35.59,27.33 31.78,31.14 22,31.14 JP8.P$8 | 36.86,23.64 38.51,25.29 38.51,30.12 37.11,31.51 34.32,31.51 JP8.P$3
HAIVE_ID2
  Top 0.61: JP9.5 61.81,69.61 59.83,67.63 55.43,67.63 54.7,66.9 54.7,56.79 | 54.7,56.79 55.97,55.52 55.97,53.1 59.78,49.29 69.56,49.29 JP12.P$8 | 54.7,56.79 53.05,55.14 53.05,50.31 53.81,49.55 53.94,49.42 54.45,48.91 57.24,48.91 JP12.P$3
HAIVE_ID3
  Top 0.61: JP13.5 69.18,10.81 71.16,12.8 75.57,12.8 76.29,13.52 76.29,23.64 | 76.29,23.64 75.02,24.91 75.02,27.33 71.21,31.14 61.43,31.14 JP16.P$8 | 76.29,23.64 77.94,25.29 77.94,30.12 76.54,31.51 73.75,31.51 JP16.P$3
HAIVE_ID4
  Top 0.61: JP17.5 101.24,69.61 99.26,67.63 94.86,67.63 94.13,66.9 94.13,56.79 | 94.13,56.79 95.4,55.52 95.4,53.1 99.21,49.29 108.99,49.29 JP20.P$8 | 94.13,56.79 92.48,55.14 92.48,50.31 93.24,49.55 93.37,49.42 93.88,48.91 96.67,48.91 JP20.P$3
HAIVE_ID5
  Top 0.61: JP21.5 108.61,10.81 110.59,12.8 114.99,12.8 115.72,13.52 115.72,23.64 | 115.72,23.64 114.45,24.91 114.45,27.33 110.64,31.14 100.86,31.14 JP24.P$8 | 115.72,23.64 117.37,25.29 117.37,30.12 115.97,31.51 113.18,31.51 JP24.P$3
HAIVE_ID6
  Top 0.61: JP25.5 140.67,69.61 138.69,67.63 134.29,67.63 133.56,66.9 133.56,56.79 | 133.56,56.79 134.83,55.52 134.83,53.1 138.64,49.29 148.42,49.29 JP28.P$8 | 133.56,56.79 131.91,55.14 131.91,50.31 132.67,49.55 132.8,49.42 133.31,48.91 136.1,48.91 JP28.P$3
HAIVE_ID7
  Top 0.61: JP29.5 148.04,10.81 150.03,12.8 154.42,12.8 155.15,13.52 155.15,23.64 | 155.15,23.64 153.88,24.91 153.88,27.33 150.07,31.14 140.29,31.14 JP32.P$8 | 155.15,23.64 156.8,25.29 156.8,30.12 155.41,31.51 152.61,31.51 JP32.P$3
HAIVE_ID8
  Top 0.61: JP33.5 180.1,69.61 178.12,67.63 173.72,67.63 172.99,66.9 172.99,56.79 | 172.99,56.79 174.26,55.52 174.26,53.1 178.07,49.29 187.85,49.29 JP36.P$8 | 172.99,56.79 171.34,55.14 171.34,50.31 172.1,49.55 172.23,49.42 172.73,48.91 175.53,48.91 JP36.P$3
HAIVE_ID9
  Top 0.61: JP37.5 187.47,10.81 189.45,12.8 193.85,12.8 194.58,13.52 194.58,23.64 | 194.58,23.64 193.31,24.91 193.31,27.33 189.5,31.14 179.72,31.14 JP40.P$8 | 194.58,23.64 196.23,25.29 196.23,30.12 194.83,31.51 192.04,31.51 JP40.P$3
HAIVE_ID10
  Top 0.61: JP41.5 22.38,137.34 20.4,135.35 16,135.35 15.27,134.63 15.27,124.51 | 15.27,124.51 16.54,123.24 16.54,120.83 20.35,117.02 30.13,117.02 JP44.P$8 | 15.27,124.51 13.62,122.86 13.62,118.04 14.38,117.27 14.51,117.15 15.02,116.64 17.81,116.64 JP44.P$3
HAIVE_ID11
  Top 0.61: JP45.5 29.75,78.54 31.73,80.52 36.13,80.52 36.86,81.25 36.86,91.37 | 36.86,91.37 35.59,92.64 35.59,95.05 31.78,98.86 22,98.86 JP48.P$8 | 36.86,91.37 38.51,93.02 38.51,97.84 37.11,99.24 34.32,99.24 JP48.P$3
HAIVE_ID12
  Top 0.61: JP49.5 61.81,137.34 59.83,135.35 55.43,135.35 54.7,134.63 54.7,124.51 | 54.7,124.51 55.97,123.24 55.97,120.83 59.78,117.02 69.56,117.02 JP52.P$8 | 54.7,124.51 53.05,122.86 53.05,118.04 53.81,117.27 53.94,117.15 54.45,116.64 57.24,116.64 JP52.P$3
HAIVE_ID13
  Top 0.61: JP53.5 69.18,78.54 71.16,80.52 75.57,80.52 76.29,81.25 76.29,91.37 | 76.29,91.37 75.02,92.64 75.02,95.05 71.21,98.86 61.43,98.86 JP56.P$8 | 76.29,91.37 77.94,93.02 77.94,97.84 76.54,99.24 73.75,99.24 JP56.P$3
HAIVE_ID14
  Top 0.61: JP57.5 101.24,137.34 99.26,135.35 94.86,135.35 94.13,134.63 94.13,124.51 | 94.13,124.51 95.4,123.24 95.4,120.83 99.21,117.02 108.99,117.02 JP60.P$8 | 94.13,124.51 92.48,122.86 92.48,118.04 93.24,117.27 93.37,117.15 93.88,116.64 96.67,116.64 JP60.P$3
HAIVE_ID15
  Top 0.61: JP61.5 108.61,78.54 110.59,80.52 114.99,80.52 115.72,81.25 115.72,91.37 | 115.72,91.37 114.45,92.64 114.45,95.05 110.64,98.86 100.86,98.86 JP64.P$8 | 115.72,91.37 117.37,93.02 117.37,97.84 115.97,99.24 113.18,99.24 JP64.P$3
HAIVE_ID16
  Top 0.61: JP65.5 140.67,137.34 138.69,135.35 134.29,135.35 133.56,134.63 133.56,124.51 | 133.56,124.51 134.83,123.24 134.83,120.83 138.64,117.02 148.42,117.02 JP68.P$8 | 133.56,124.51 131.91,122.86 131.91,118.04 132.67,117.27 132.8,117.15 133.31,116.64 136.1,116.64 JP68.P$3
HAIVE_ID17
  Top 0.61: JP69.5 148.04,78.54 150.03,80.52 154.42,80.52 155.15,81.25 155.15,91.37 | 155.15,91.37 153.88,92.64 153.88,95.05 150.07,98.86 140.29,98.86 JP72.P$8 | 155.15,91.37 156.8,93.02 156.8,97.84 155.41,99.24 152.61,99.24 JP72.P$3
HAIVE_ID18
  Top 0.61: JP73.5 180.1,137.34 178.12,135.35 173.72,135.35 172.99,134.63 172.99,124.51 | 172.99,124.51 174.26,123.24 174.26,120.83 178.07,117.02 187.85,117.02 JP76.P$8 | 172.99,124.51 171.34,122.86 171.34,118.04 172.1,117.27 172.23,117.15 172.73,116.64 175.53,116.64 JP76.P$3
HAIVE_ID19
  Top 0.61: JP77.5 187.47,78.54 189.45,80.52 193.85,80.52 194.58,81.25 194.58,91.37 | 194.58,91.37 193.31,92.64 193.31,95.05 189.5,98.86 179.72,98.86 JP80.P$8 | 194.58,91.37 196.23,93.02 196.23,97.84 194.83,99.24 192.04,99.24 JP80.P$3
SLOT_ID
  Top 0.61: JP1.4 19.84,71 17.83,68.98 13.5,68.98 11.46,66.95 11.46,51.71 | 11.46,51.71 10.19,50.44 10.19,47.9 12.83,45.26 35.74,45.26 JP4.P$10 | 11.46,51.71 12.22,50.95 12.22,49.42 JP4.P$1
SLOT_ID1
  Top 0.61: JP5.4 34.3,11.45 38.63,11.45 40.67,13.48 40.67,28.72 | 40.67,28.72 41.94,29.99 41.94,32.53 39.3,35.17 16.38,35.17 JP8.P$10 | 40.67,28.72 39.91,29.48 39.91,31.01 JP8.P$1
SLOT_ID2
  Top 0.61: JP9.4 59.27,71 57.26,68.98 52.93,68.98 50.89,66.95 50.89,51.71 | 50.89,51.71 49.62,50.44 49.62,47.9 52.26,45.26 75.18,45.26 JP12.P$10 | 50.89,51.71 51.65,50.95 51.65,49.42 JP12.P$1
SLOT_ID3
  Top 0.61: JP13.4 73.73,11.45 78.07,11.45 80.1,13.48 80.1,28.72 | 80.1,28.72 81.37,29.99 81.37,32.53 78.73,35.17 55.82,35.17 JP16.P$10 | 80.1,28.72 79.34,29.48 79.34,31.01 JP16.P$1
SLOT_ID4
  Top 0.61: JP17.4 98.7,71 96.69,68.98 92.35,68.98 90.32,66.95 90.32,51.71 | 90.32,51.71 89.05,50.44 89.05,47.9 91.69,45.26 114.6,45.26 JP20.P$10 | 90.32,51.71 91.08,50.95 91.08,49.42 JP20.P$1
SLOT_ID5
  Top 0.61: JP21.4 113.16,11.45 117.49,11.45 119.53,13.48 119.53,28.72 | 119.53,28.72 120.8,29.99 120.8,32.53 118.16,35.17 95.24,35.17 JP24.P$10 | 119.53,28.72 118.77,29.48 118.77,31.01 JP24.P$1
SLOT_ID6
  Top 0.61: JP25.4 138.13,71 136.12,68.98 131.79,68.98 129.75,66.95 129.75,51.71 | 129.75,51.71 128.48,50.44 128.48,47.9 131.12,45.26 154.04,45.26 JP28.P$10 | 129.75,51.71 130.51,50.95 130.51,49.42 JP28.P$1
SLOT_ID7
  Top 0.61: JP29.4 152.59,11.45 156.93,11.45 158.96,13.48 158.96,28.72 | 158.96,28.72 160.23,29.99 160.23,32.53 157.59,35.17 134.68,35.17 JP32.P$10 | 158.96,28.72 158.2,29.48 158.2,31.01 JP32.P$1
SLOT_ID8
  Top 0.61: JP33.4 177.56,71 175.55,68.98 171.21,68.98 169.18,66.95 169.18,51.71 | 169.18,51.71 167.91,50.44 167.91,47.9 170.55,45.26 193.46,45.26 JP36.P$10 | 169.18,51.71 169.94,50.95 169.94,49.42 JP36.P$1
SLOT_ID9
  Top 0.61: JP37.4 192.02,11.45 196.35,11.45 198.39,13.48 198.39,28.72 | 198.39,28.72 199.66,29.99 199.66,32.53 197.02,35.17 174.1,35.17 JP40.P$10 | 198.39,28.72 197.63,29.48 197.63,31.01 JP40.P$1
SLOT_ID10
  Top 0.61: JP41.4 19.84,138.72 17.83,136.71 13.5,136.71 11.46,134.67 11.46,119.43 | 11.46,119.43 10.19,118.16 10.19,115.62 12.83,112.98 35.74,112.98 JP44.P$10 | 11.46,119.43 12.22,118.67 12.22,117.15 JP44.P$1
SLOT_ID11
  Top 0.61: JP45.4 32.29,77.16 34.3,79.17 38.63,79.17 40.67,81.21 40.67,96.45 | 40.67,96.45 41.94,97.72 41.94,100.26 39.3,102.89 16.38,102.89 JP48.P$10 | 40.67,96.45 39.91,97.21 39.91,98.73 JP48.P$1
SLOT_ID12
  Top 0.61: JP49.4 59.27,138.72 57.26,136.71 52.93,136.71 50.89,134.67 50.89,119.43 | 50.89,119.43 49.62,118.16 49.62,115.62 52.26,112.98 75.18,112.98 JP52.P$10 | 50.89,119.43 51.65,118.67 51.65,117.15 JP52.P$1
SLOT_ID13
  Top 0.61: JP53.4 71.72,77.16 73.73,79.17 78.07,79.17 80.1,81.21 80.1,96.45 | 80.1,96.45 81.37,97.72 81.37,100.26 78.73,102.89 55.82,102.89 JP56.P$10 | 80.1,96.45 79.34,97.21 79.34,98.73 JP56.P$1
SLOT_ID14
  Top 0.61: JP57.4 98.7,138.72 96.69,136.71 92.35,136.71 90.32,134.67 90.32,119.43 | 90.32,119.43 89.05,118.16 89.05,115.62 91.69,112.98 114.6,112.98 JP60.P$10 | 90.32,119.43 91.08,118.67 91.08,117.15 JP60.P$1
SLOT_ID15
  Top 0.61: JP61.4 111.15,77.16 113.16,79.17 117.49,79.17 119.53,81.21 119.53,96.45 | 119.53,96.45 120.8,97.72 120.8,100.26 118.16,102.89 95.24,102.89 JP64.P$10 | 119.53,96.45 118.77,97.21 118.77,98.73 JP64.P$1
SLOT_ID16
  Top 0.61: JP65.4 138.13,138.72 136.12,136.71 131.79,136.71 129.75,134.67 129.75,119.43 | 129.75,119.43 128.48,118.16 128.48,115.62 131.12,112.98 154.04,112.98 JP68.P$10 | 129.75,119.43 130.51,118.67 130.51,117.15 JP68.P$1
SLOT_ID17
  Top 0.61: JP69.4 150.58,77.16 152.59,79.17 156.93,79.17 158.96,81.21 158.96,96.45 | 158.96,96.45 160.23,97.72 160.23,100.26 157.59,102.89 134.68,102.89 JP72.P$10 | 158.96,96.45 158.2,97.21 158.2,98.73 JP72.P$1
SLOT_ID18
  Top 0.61: JP73.4 177.56,138.72 175.55,136.71 171.21,136.71 169.18,134.67 169.18,119.43 | 169.18,119.43 167.91,118.16 167.91,115.62 170.55,112.98 193.46,112.98 JP76.P$10 | 169.18,119.43 169.94,118.67 169.94,117.15 JP76.P$1
SLOT_ID19
  Top 0.61: JP77.4 190.01,77.16 192.02,79.17 196.35,79.17 198.39,81.21 198.39,96.45 | 198.39,96.45 199.66,97.72 199.66,100.26 197.02,102.89 174.1,102.89 JP80.P$10 | 198.39,96.45 197.63,97.21 197.63,98.73 JP80.P$1

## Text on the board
tPlace: Pololu_#2855 | Pololu_#2855 | Pololu_#2855 | Pololu_#2855 | Pololu_#2855 | Pololu_#2855 | Pololu_#2855 | Pololu_#2855 | Pololu_#2855 | Pololu_#2855 | Pololu_#2855 | Pololu_#2855 | Pololu_#2855 | Pololu_#2855 | Pololu_#2855 | Pololu_#2855 | Pololu_#2855 | Pololu_#2855 | Pololu_#2855 | Pololu_#2855
Milling: v-score | v-score | v-score | v-score | v-score | v-score | v-score | v-score | v-score | v-score | v-score
_tNames: JP1 | JP1 | JP1 | JP1 | JP1 | JP2 | JP2 | JP2 | JP2 | JP2 | JP3 | JP3 | JP3 | JP3 | JP3 | JP4 | JP4 | JP4 | JP4 | JP4 | JP4 | JP4 | JP4 | JP4 | JP4 | JP3 | JP3 | JP3 | JP3 | JP3 | JP2 | JP2 | JP2 | JP2 | JP2 | JP1 | JP1 | JP1 | JP1 | JP1 | JP1 | JP1 | JP1 | JP1 | JP1 | JP2 | JP2 | JP2 | JP2 | JP2 | JP3 | JP3 | JP3 | JP3 | JP3 | JP4 | JP4 | JP4 | JP4 | JP4 | JP4 | JP4 | JP4 | JP4 | JP4 | JP3 | JP3 | JP3 | JP3 | JP3 | JP2 | JP2 | JP2 | JP2 | JP2 | JP1 | JP1 | JP1 | JP1 | JP1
